FUNCTION_BLOCK FB 1004
TITLE =FB_SCTMi_IOL
//(*//////////////////////////////////////////////////////////////////////////////
////------------------------------------------------------------------------------
//// Copyright (C) - J. Schmalz GmbH 2018 - All Rights Reserved
//// Subject to change without notice
////------------------------------------------------------------------------------
//// This function block controls a Schmalz SCTMi with IO-Link interface via the
//// process data. With this function block all possible combinations of ejectors
//// can be controlled.
//// Further information can be found in the funktionblock documentation.
////------------------------------------------------------------------------------
//// Version:       1.0
//// Issue DATE:    2018-07-20
////------------------------------------------------------------------------------
////////////////////////////////////////////////////////////////////////////////*)

VERSION : 0.0


VAR_INPUT
  iInputPressure : INT ;
  bVacOnEjector1 : BOOL ;
  bBlowOffEjector1 : BOOL ;
  bVacOnEjector2 : BOOL ;
  bBlowOffEjector2 : BOOL ;
  bVacOnEjector3 : BOOL ;
  bBlowOffEjector3 : BOOL ;
  bVacOnEjector4 : BOOL ;
  bBlowOffEjector4 : BOOL ;
  bVacOnEjector5 : BOOL ;
  bBlowOffEjector5 : BOOL ;
  bVacOnEjector6 : BOOL ;
  bBlowOffEjector6 : BOOL ;
  bVacOnEjector7 : BOOL ;
  bBlowOffEjector7 : BOOL ;
  bVacOnEjector8 : BOOL ;
  bBlowOffEjector8 : BOOL ;
  bVacOnEjector9 : BOOL ;
  bBlowOffEjector9 : BOOL ;
  bVacOnEjector10 : BOOL ;
  bBlowOffEjector10 : BOOL ;
  bVacOnEjector11 : BOOL ;
  bBlowOffEjector11 : BOOL ;
  bVacOnEjector12 : BOOL ;
  bBlowOffEjector12 : BOOL ;
  bVacOnEjector13 : BOOL ;
  bBlowOffEjector13 : BOOL ;
  bVacOnEjector14 : BOOL ;
  bBlowOffEjector14 : BOOL ;
  bVacOnEjector15 : BOOL ;
  bBlowOffEjector15 : BOOL ;
  bVacOnEjector16 : BOOL ;
  bBlowOffEjector16 : BOOL ;
  iNumberOfEjectors : INT ;
  iValveTypes : INT ;
  btPDIData0 : BYTE ;
  btPDIData1 : BYTE ;
  btPDIData2 : BYTE ;
  btPDIData3 : BYTE ;
  btPDIData4 : BYTE ;
  btPDIData5 : BYTE ;
  btPDIData6 : BYTE ;
  btPDIData7 : BYTE ;
END_VAR
VAR_OUTPUT
  bDeviceStateGreen : BOOL ;
  bDeviceStateYellow : BOOL ;
  bDeviceStateOrange : BOOL ;
  bDeviceStateRed : BOOL ;
  btErrorByteCU : BYTE ;
  btWarningByteCU : BYTE ;
  wPrimSupplyVoltageCU : WORD ;
  wAuxSupplyVoltageCU : WORD ;
  wTotalAirConsCU : WORD ;
  stDataEjector1 : STRUCT
   btErrorByte : BYTE ;
   btWarningByte : BYTE ;
   btLeakageOfLastCycle : BYTE ;
   wSystemVacuum : WORD ;
   wEvacuationTimeT1 : WORD ;
   wLastFreeFlowVacuum : WORD ;
   wAirConsumptionOfLastCyc : WORD ;
   bAirSavingFunktion_H1 : BOOL ;
   bPartPresent_H2 : BOOL ;
  END_STRUCT ;
  stDataEjector2 : STRUCT
   btErrorByte : BYTE ;
   btWarningByte : BYTE ;
   btLeakageOfLastCycle : BYTE ;
   wSystemVacuum : WORD ;
   wEvacuationTimeT1 : WORD ;
   wLastFreeFlowVacuum : WORD ;
   wAirConsumptionOfLastCyc : WORD ;
   bAirSavingFunktion_H1 : BOOL ;
   bPartPresent_H2 : BOOL ;
  END_STRUCT ;
  stDataEjector3 : STRUCT
   btErrorByte : BYTE ;
   btWarningByte : BYTE ;
   btLeakageOfLastCycle : BYTE ;
   wSystemVacuum : WORD ;
   wEvacuationTimeT1 : WORD ;
   wLastFreeFlowVacuum : WORD ;
   wAirConsumptionOfLastCyc : WORD ;
   bAirSavingFunktion_H1 : BOOL ;
   bPartPresent_H2 : BOOL ;
  END_STRUCT ;
  stDataEjector4 : STRUCT
   btErrorByte : BYTE ;
   btWarningByte : BYTE ;
   btLeakageOfLastCycle : BYTE ;
   wSystemVacuum : WORD ;
   wEvacuationTimeT1 : WORD ;
   wLastFreeFlowVacuum : WORD ;
   wAirConsumptionOfLastCyc : WORD ;
   bAirSavingFunktion_H1 : BOOL ;
   bPartPresent_H2 : BOOL ;
  END_STRUCT ;
  stDataEjector5 : STRUCT
   btErrorByte : BYTE ;
   btWarningByte : BYTE ;
   btLeakageOfLastCycle : BYTE ;
   wSystemVacuum : WORD ;
   wEvacuationTimeT1 : WORD ;
   wLastFreeFlowVacuum : WORD ;
   wAirConsumptionOfLastCyc : WORD ;
   bAirSavingFunktion_H1 : BOOL ;
   bPartPresent_H2 : BOOL ;
  END_STRUCT ;
  stDataEjector6 : STRUCT
   btErrorByte : BYTE ;
   btWarningByte : BYTE ;
   btLeakageOfLastCycle : BYTE ;
   wSystemVacuum : WORD ;
   wEvacuationTimeT1 : WORD ;
   wLastFreeFlowVacuum : WORD ;
   wAirConsumptionOfLastCyc : WORD ;
   bAirSavingFunktion_H1 : BOOL ;
   bPartPresent_H2 : BOOL ;
  END_STRUCT ;
  stDataEjector7 : STRUCT
   btErrorByte : BYTE ;
   btWarningByte : BYTE ;
   btLeakageOfLastCycle : BYTE ;
   wSystemVacuum : WORD ;
   wEvacuationTimeT1 : WORD ;
   wLastFreeFlowVacuum : WORD ;
   wAirConsumptionOfLastCyc : WORD ;
   bAirSavingFunktion_H1 : BOOL ;
   bPartPresent_H2 : BOOL ;
  END_STRUCT ;
  stDataEjector8 : STRUCT
   btErrorByte : BYTE ;
   btWarningByte : BYTE ;
   btLeakageOfLastCycle : BYTE ;
   wSystemVacuum : WORD ;
   wEvacuationTimeT1 : WORD ;
   wLastFreeFlowVacuum : WORD ;
   wAirConsumptionOfLastCyc : WORD ;
   bAirSavingFunktion_H1 : BOOL ;
   bPartPresent_H2 : BOOL ;
  END_STRUCT ;
  stDataEjector9 : STRUCT
   btErrorByte : BYTE ;
   btWarningByte : BYTE ;
   btLeakageOfLastCycle : BYTE ;
   wSystemVacuum : WORD ;
   wEvacuationTimeT1 : WORD ;
   wLastFreeFlowVacuum : WORD ;
   wAirConsumptionOfLastCyc : WORD ;
   bAirSavingFunktion_H1 : BOOL ;
   bPartPresent_H2 : BOOL ;
  END_STRUCT ;
  stDataEjector10 : STRUCT
   btErrorByte : BYTE ;
   btWarningByte : BYTE ;
   btLeakageOfLastCycle : BYTE ;
   wSystemVacuum : WORD ;
   wEvacuationTimeT1 : WORD ;
   wLastFreeFlowVacuum : WORD ;
   wAirConsumptionOfLastCyc : WORD ;
   bAirSavingFunktion_H1 : BOOL ;
   bPartPresent_H2 : BOOL ;
  END_STRUCT ;
  stDataEjector11 : STRUCT
   btErrorByte : BYTE ;
   btWarningByte : BYTE ;
   btLeakageOfLastCycle : BYTE ;
   wSystemVacuum : WORD ;
   wEvacuationTimeT1 : WORD ;
   wLastFreeFlowVacuum : WORD ;
   wAirConsumptionOfLastCyc : WORD ;
   bAirSavingFunktion_H1 : BOOL ;
   bPartPresent_H2 : BOOL ;
  END_STRUCT ;
  stDataEjector12 : STRUCT
   btErrorByte : BYTE ;
   btWarningByte : BYTE ;
   btLeakageOfLastCycle : BYTE ;
   wSystemVacuum : WORD ;
   wEvacuationTimeT1 : WORD ;
   wLastFreeFlowVacuum : WORD ;
   wAirConsumptionOfLastCyc : WORD ;
   bAirSavingFunktion_H1 : BOOL ;
   bPartPresent_H2 : BOOL ;
  END_STRUCT ;
  stDataEjector13 : STRUCT
   btErrorByte : BYTE ;
   btWarningByte : BYTE ;
   btLeakageOfLastCycle : BYTE ;
   wSystemVacuum : WORD ;
   wEvacuationTimeT1 : WORD ;
   wLastFreeFlowVacuum : WORD ;
   wAirConsumptionOfLastCyc : WORD ;
   bAirSavingFunktion_H1 : BOOL ;
   bPartPresent_H2 : BOOL ;
  END_STRUCT ;
  stDataEjector14 : STRUCT
   btErrorByte : BYTE ;
   btWarningByte : BYTE ;
   btLeakageOfLastCycle : BYTE ;
   wSystemVacuum : WORD ;
   wEvacuationTimeT1 : WORD ;
   wLastFreeFlowVacuum : WORD ;
   wAirConsumptionOfLastCyc : WORD ;
   bAirSavingFunktion_H1 : BOOL ;
   bPartPresent_H2 : BOOL ;
  END_STRUCT ;
  stDataEjector15 : STRUCT
   btErrorByte : BYTE ;
   btWarningByte : BYTE ;
   btLeakageOfLastCycle : BYTE ;
   wSystemVacuum : WORD ;
   wEvacuationTimeT1 : WORD ;
   wLastFreeFlowVacuum : WORD ;
   wAirConsumptionOfLastCyc : WORD ;
   bAirSavingFunktion_H1 : BOOL ;
   bPartPresent_H2 : BOOL ;
  END_STRUCT ;
  stDataEjector16 : STRUCT
   btErrorByte : BYTE ;
   btWarningByte : BYTE ;
   btLeakageOfLastCycle : BYTE ;
   wSystemVacuum : WORD ;
   wEvacuationTimeT1 : WORD ;
   wLastFreeFlowVacuum : WORD ;
   wAirConsumptionOfLastCyc : WORD ;
   bAirSavingFunktion_H1 : BOOL ;
   bPartPresent_H2 : BOOL ;
  END_STRUCT ;
  btPDOData0 : BYTE ;
  btPDOData1 : BYTE ;
  btPDOData2 : BYTE ;
  btPDOData3 : BYTE ;
  btPDOData4 : BYTE ;
  btPDOData5 : BYTE ;
END_VAR
VAR
  iStep : INT ;
END_VAR
BEGIN
NETWORK
TITLE =SCL Netzwerk
//generiert vom SCL Übersetzer Version:  SCLCOMP K05.06.00.00_11.01.00.01 release
      SET   ;
      SAVE  ;
      =     L      0.1;
      L     #iStep;
      L     0;
      TAK   ;
      ==I   ;
      T     LW     2;
      SPB   A7d1;
      SPA   A7d2;
A7d1: CLR   ;
      =     DIX [AR2,P#252.0];
      =     DIX [AR2,P#252.1];
      =     DIX [AR2,P#252.2];
      =     DIX [AR2,P#252.3];
      =     DIX [AR2,P#252.4];
      =     DIX [AR2,P#252.6];
      =     DIX [AR2,P#252.7];
      U     DIX [AR2,P#10.5];
      NOT   ;
      SPBN  A7d0;
      L     #btPDIData1;
      T     #btErrorByteCU;
      L     #btPDIData3;
      T     DIB [AR2,P#22.0];
      L     #btPDIData2;
      T     DIB [AR2,P#23.0];
      L     #iStep;
      L     1;
      +I    ;
      T     #iStep;
      SPA   A7d0;
A7d2: L     1;
      L     LW     2;
      ==I   ;
      SPB   A7d4;
      SPA   A7d5;
A7d4: SET   ;
      =     DIX [AR2,P#252.6];
      CLR   ;
      =     DIX [AR2,P#252.7];
      U     DIX [AR2,P#10.5];
      SPBN  A7d0;
      L     #btPDIData1;
      T     #btWarningByteCU;
      L     #btPDIData3;
      T     DIB [AR2,P#24.0];
      L     #btPDIData2;
      T     DIB [AR2,P#25.0];
      L     #iStep;
      L     1;
      +I    ;
      T     #iStep;
      SPA   A7d0;
A7d5: L     2;
      L     LW     2;
      ==I   ;
      SPB   A7d7;
      SPA   A7d8;
A7d7: CLR   ;
      =     DIX [AR2,P#252.6];
      =     DIX [AR2,P#252.7];
      U     DIX [AR2,P#10.5];
      NOT   ;
      SPBN  A7d0;
      L     #iStep;
      L     1;
      +I    ;
      T     #iStep;
      SPA   A7d0;
A7d8: L     3;
      L     LW     2;
      ==I   ;
      SPB   A7da;
      SPA   A7db;
A7da: CLR   ;
      =     DIX [AR2,P#252.6];
      SET   ;
      =     DIX [AR2,P#252.7];
      U     DIX [AR2,P#10.5];
      SPBN  A7d0;
      L     #iStep;
      L     1;
      +I    ;
      T     #iStep;
      SPA   A7d0;
A7db: L     4;
      L     LW     2;
      ==I   ;
      SPB   A7dd;
      SPA   A7de;
A7dd: CLR   ;
      =     DIX [AR2,P#252.6];
      =     DIX [AR2,P#252.7];
      U     DIX [AR2,P#10.5];
      NOT   ;
      SPBN  A7d0;
      L     #iStep;
      L     1;
      +I    ;
      T     #iStep;
      SPA   A7d0;
A7de: L     5;
      L     LW     2;
      ==I   ;
      SPB   A7e0;
      SPA   A7e1;
A7e0: SET   ;
      =     DIX [AR2,P#252.6];
      =     DIX [AR2,P#252.7];
      U     DIX [AR2,P#10.5];
      SPBN  A7d0;
      L     #btPDIData3;
      T     DIB [AR2,P#26.0];
      L     #btPDIData2;
      T     DIB [AR2,P#27.0];
      L     #iStep;
      L     1;
      +I    ;
      T     #iStep;
      SPA   A7d0;
A7e1: L     6;
      L     LW     2;
      ==I   ;
      SPB   A7e3;
      SPA   A7e4;
A7e3: L     #iNumberOfEjectors;
      L     1;
      >=I   ;
      SPBN  A7e5;
      L     #iStep;
      +I    ;
      T     #iStep;
      SPA   A7d0;
A7e5: L     0;
      T     #iStep;
      SPA   A7d0;
A7e4: L     7;
      L     LW     2;
      ==I   ;
      SPB   A7e7;
      SPA   A7e8;
A7e7: SET   ;
      =     DIX [AR2,P#252.0];
      CLR   ;
      =     DIX [AR2,P#252.1];
      =     DIX [AR2,P#252.2];
      =     DIX [AR2,P#252.3];
      =     DIX [AR2,P#252.4];
      =     DIX [AR2,P#252.6];
      =     DIX [AR2,P#252.7];
      U     DIX [AR2,P#10.5];
      NOT   ;
      SPBN  A7d0;
      L     #btPDIData1;
      T     #stDataEjector1.btErrorByte;
      L     #btPDIData2;
      UD    DW#16#FF;
      L     8;
      TAK   ;
      LAR1  ;
      TAK   ;
      L     DW#16#10;
      >=I   ;
      SPB   I007;
      TAK   ;
      TAR1  ;
      SLW   ;
      SPA   I008;
I007: L     DW#16#0;
I008: UD    DW#16#FFFF;
      L     #btPDIData3;
      UD    DW#16#FF;
      OW    ;
      T     #stDataEjector1.wSystemVacuum;
      L     #iStep;
      L     1;
      +I    ;
      T     #iStep;
      SPA   A7d0;
A7e8: L     8;
      L     LW     2;
      ==I   ;
      SPB   A7ea;
      SPA   A7eb;
A7ea: SET   ;
      =     DIX [AR2,P#252.6];
      CLR   ;
      =     DIX [AR2,P#252.7];
      U     DIX [AR2,P#10.5];
      SPBN  A7d0;
      L     #btPDIData1;
      T     #stDataEjector1.btWarningByte;
      L     #btPDIData2;
      UD    DW#16#FF;
      L     8;
      TAK   ;
      LAR1  ;
      TAK   ;
      L     DW#16#10;
      >=I   ;
      SPB   I009;
      TAK   ;
      TAR1  ;
      SLW   ;
      SPA   I00a;
I009: L     DW#16#0;
I00a: UD    DW#16#FFFF;
      L     #btPDIData3;
      UD    DW#16#FF;
      OW    ;
      T     #stDataEjector1.wEvacuationTimeT1;
      L     #iStep;
      L     1;
      +I    ;
      T     #iStep;
      SPA   A7d0;
A7eb: L     9;
      L     LW     2;
      ==I   ;
      SPB   A7ed;
      SPA   A7ee;
A7ed: CLR   ;
      =     DIX [AR2,P#252.6];
      =     DIX [AR2,P#252.7];
      U     DIX [AR2,P#10.5];
      NOT   ;
      SPBN  A7d0;
      L     #iStep;
      L     1;
      +I    ;
      T     #iStep;
      SPA   A7d0;
A7ee: L     10;
      L     LW     2;
      ==I   ;
      SPB   A7f0;
      SPA   A7f1;
A7f0: CLR   ;
      =     DIX [AR2,P#252.6];
      SET   ;
      =     DIX [AR2,P#252.7];
      U     DIX [AR2,P#10.5];
      SPBN  A7d0;
      L     #btPDIData2;
      UD    DW#16#FF;
      L     8;
      TAK   ;
      LAR1  ;
      TAK   ;
      L     DW#16#10;
      >=I   ;
      SPB   I00b;
      TAK   ;
      TAR1  ;
      SLW   ;
      SPA   I00c;
I00b: L     DW#16#0;
I00c: UD    DW#16#FFFF;
      L     #btPDIData3;
      UD    DW#16#FF;
      OW    ;
      T     #stDataEjector1.wLastFreeFlowVacuum;
      L     #iStep;
      L     1;
      +I    ;
      T     #iStep;
      SPA   A7d0;
A7f1: L     11;
      L     LW     2;
      ==I   ;
      SPB   A7f3;
      SPA   A7f4;
A7f3: CLR   ;
      =     DIX [AR2,P#252.6];
      =     DIX [AR2,P#252.7];
      U     DIX [AR2,P#10.5];
      NOT   ;
      SPBN  A7d0;
      L     #iStep;
      L     1;
      +I    ;
      T     #iStep;
      SPA   A7d0;
A7f4: L     12;
      L     LW     2;
      ==I   ;
      SPB   A7f6;
      SPA   A7f7;
A7f6: SET   ;
      =     DIX [AR2,P#252.6];
      =     DIX [AR2,P#252.7];
      U     DIX [AR2,P#10.5];
      SPBN  A7d0;
      L     #btPDIData1;
      T     #stDataEjector1.btLeakageOfLastCycle;
      L     #btPDIData2;
      UD    DW#16#FF;
      L     8;
      TAK   ;
      LAR1  ;
      TAK   ;
      L     DW#16#10;
      >=I   ;
      SPB   I00d;
      TAK   ;
      TAR1  ;
      SLW   ;
      SPA   I00e;
I00d: L     DW#16#0;
I00e: UD    DW#16#FFFF;
      L     #btPDIData3;
      UD    DW#16#FF;
      OW    ;
      T     #stDataEjector1.wAirConsumptionOfLastCyc;
      L     #iStep;
      L     1;
      +I    ;
      T     #iStep;
      SPA   A7d0;
A7f7: L     13;
      L     LW     2;
      ==I   ;
      SPB   A7f9;
      SPA   A7fa;
A7f9: L     #iNumberOfEjectors;
      L     2;
      >=I   ;
      SPBN  A7fb;
      L     #iStep;
      L     1;
      +I    ;
      T     #iStep;
      SPA   A7d0;
A7fb: L     0;
      T     #iStep;
      SPA   A7d0;
A7fa: L     14;
      L     LW     2;
      ==I   ;
      SPB   A7fd;
      SPA   A7fe;
A7fd: CLR   ;
      =     DIX [AR2,P#252.0];
      SET   ;
      =     DIX [AR2,P#252.1];
      CLR   ;
      =     DIX [AR2,P#252.2];
      =     DIX [AR2,P#252.3];
      =     DIX [AR2,P#252.4];
      =     DIX [AR2,P#252.6];
      =     DIX [AR2,P#252.7];
      U     DIX [AR2,P#10.5];
      NOT   ;
      SPBN  A7d0;
      L     #btPDIData1;
      T     #stDataEjector2.btErrorByte;
      L     #btPDIData2;
      UD    DW#16#FF;
      L     8;
      TAK   ;
      LAR1  ;
      TAK   ;
      L     DW#16#10;
      >=I   ;
      SPB   I00f;
      TAK   ;
      TAR1  ;
      SLW   ;
      SPA   I010;
I00f: L     DW#16#0;
I010: UD    DW#16#FFFF;
      L     #btPDIData3;
      UD    DW#16#FF;
      OW    ;
      T     #stDataEjector2.wSystemVacuum;
      L     #iStep;
      L     1;
      +I    ;
      T     #iStep;
      SPA   A7d0;
A7fe: L     15;
      L     LW     2;
      ==I   ;
      SPB   A800;
      SPA   A801;
A800: SET   ;
      =     DIX [AR2,P#252.6];
      CLR   ;
      =     DIX [AR2,P#252.7];
      U     DIX [AR2,P#10.5];
      SPBN  A7d0;
      L     #btPDIData1;
      T     #stDataEjector2.btWarningByte;
      L     #btPDIData2;
      UD    DW#16#FF;
      L     8;
      TAK   ;
      LAR1  ;
      TAK   ;
      L     DW#16#10;
      >=I   ;
      SPB   I011;
      TAK   ;
      TAR1  ;
      SLW   ;
      SPA   I012;
I011: L     DW#16#0;
I012: UD    DW#16#FFFF;
      L     #btPDIData3;
      UD    DW#16#FF;
      OW    ;
      T     #stDataEjector2.wEvacuationTimeT1;
      L     #iStep;
      L     1;
      +I    ;
      T     #iStep;
      SPA   A7d0;
A801: L     16;
      L     LW     2;
      ==I   ;
      SPB   A803;
      SPA   A804;
A803: CLR   ;
      =     DIX [AR2,P#252.6];
      =     DIX [AR2,P#252.7];
      U     DIX [AR2,P#10.5];
      NOT   ;
      SPBN  A7d0;
      L     #iStep;
      L     1;
      +I    ;
      T     #iStep;
      SPA   A7d0;
A804: L     17;
      L     LW     2;
      ==I   ;
      SPB   A806;
      SPA   A807;
A806: CLR   ;
      =     DIX [AR2,P#252.6];
      SET   ;
      =     DIX [AR2,P#252.7];
      U     DIX [AR2,P#10.5];
      SPBN  A7d0;
      L     #btPDIData2;
      UD    DW#16#FF;
      L     8;
      TAK   ;
      LAR1  ;
      TAK   ;
      L     DW#16#10;
      >=I   ;
      SPB   I013;
      TAK   ;
      TAR1  ;
      SLW   ;
      SPA   I014;
I013: L     DW#16#0;
I014: UD    DW#16#FFFF;
      L     #btPDIData3;
      UD    DW#16#FF;
      OW    ;
      T     #stDataEjector2.wLastFreeFlowVacuum;
      L     #iStep;
      L     1;
      +I    ;
      T     #iStep;
      SPA   A7d0;
A807: L     18;
      L     LW     2;
      ==I   ;
      SPB   A809;
      SPA   A80a;
A809: CLR   ;
      =     DIX [AR2,P#252.6];
      =     DIX [AR2,P#252.7];
      U     DIX [AR2,P#10.5];
      NOT   ;
      SPBN  A7d0;
      L     #iStep;
      L     1;
      +I    ;
      T     #iStep;
      SPA   A7d0;
A80a: L     19;
      L     LW     2;
      ==I   ;
      SPB   A80c;
      SPA   A80d;
A80c: SET   ;
      =     DIX [AR2,P#252.6];
      =     DIX [AR2,P#252.7];
      U     DIX [AR2,P#10.5];
      SPBN  A7d0;
      L     #btPDIData1;
      T     #stDataEjector2.btLeakageOfLastCycle;
      L     #btPDIData2;
      UD    DW#16#FF;
      L     8;
      TAK   ;
      LAR1  ;
      TAK   ;
      L     DW#16#10;
      >=I   ;
      SPB   I015;
      TAK   ;
      TAR1  ;
      SLW   ;
      SPA   I016;
I015: L     DW#16#0;
I016: UD    DW#16#FFFF;
      L     #btPDIData3;
      UD    DW#16#FF;
      OW    ;
      T     #stDataEjector2.wAirConsumptionOfLastCyc;
      L     #iStep;
      L     1;
      +I    ;
      T     #iStep;
      SPA   A7d0;
A80d: L     20;
      L     LW     2;
      ==I   ;
      SPB   A80f;
      SPA   A810;
A80f: L     #iNumberOfEjectors;
      L     3;
      >=I   ;
      SPBN  A811;
      L     #iStep;
      L     1;
      +I    ;
      T     #iStep;
      SPA   A7d0;
A811: L     0;
      T     #iStep;
      SPA   A7d0;
A810: L     21;
      L     LW     2;
      ==I   ;
      SPB   A813;
      SPA   A814;
A813: SET   ;
      =     DIX [AR2,P#252.0];
      =     DIX [AR2,P#252.1];
      CLR   ;
      =     DIX [AR2,P#252.2];
      =     DIX [AR2,P#252.3];
      =     DIX [AR2,P#252.4];
      =     DIX [AR2,P#252.6];
      =     DIX [AR2,P#252.7];
      U     DIX [AR2,P#10.5];
      NOT   ;
      SPBN  A7d0;
      L     #btPDIData1;
      T     #stDataEjector3.btErrorByte;
      L     #btPDIData2;
      UD    DW#16#FF;
      L     8;
      TAK   ;
      LAR1  ;
      TAK   ;
      L     DW#16#10;
      >=I   ;
      SPB   I017;
      TAK   ;
      TAR1  ;
      SLW   ;
      SPA   I018;
I017: L     DW#16#0;
I018: UD    DW#16#FFFF;
      L     #btPDIData3;
      UD    DW#16#FF;
      OW    ;
      T     #stDataEjector3.wSystemVacuum;
      L     #iStep;
      L     1;
      +I    ;
      T     #iStep;
      SPA   A7d0;
A814: L     22;
      L     LW     2;
      ==I   ;
      SPB   A816;
      SPA   A817;
A816: SET   ;
      =     DIX [AR2,P#252.6];
      CLR   ;
      =     DIX [AR2,P#252.7];
      U     DIX [AR2,P#10.5];
      SPBN  A7d0;
      L     #btPDIData1;
      T     #stDataEjector3.btWarningByte;
      L     #btPDIData2;
      UD    DW#16#FF;
      L     8;
      TAK   ;
      LAR1  ;
      TAK   ;
      L     DW#16#10;
      >=I   ;
      SPB   I019;
      TAK   ;
      TAR1  ;
      SLW   ;
      SPA   I01a;
I019: L     DW#16#0;
I01a: UD    DW#16#FFFF;
      L     #btPDIData3;
      UD    DW#16#FF;
      OW    ;
      T     #stDataEjector3.wEvacuationTimeT1;
      L     #iStep;
      L     1;
      +I    ;
      T     #iStep;
      SPA   A7d0;
A817: L     23;
      L     LW     2;
      ==I   ;
      SPB   A819;
      SPA   A81a;
A819: CLR   ;
      =     DIX [AR2,P#252.6];
      =     DIX [AR2,P#252.7];
      U     DIX [AR2,P#10.5];
      NOT   ;
      SPBN  A7d0;
      L     #iStep;
      L     1;
      +I    ;
      T     #iStep;
      SPA   A7d0;
A81a: L     24;
      L     LW     2;
      ==I   ;
      SPB   A81c;
      SPA   A81d;
A81c: CLR   ;
      =     DIX [AR2,P#252.6];
      SET   ;
      =     DIX [AR2,P#252.7];
      U     DIX [AR2,P#10.5];
      SPBN  A7d0;
      L     #btPDIData2;
      UD    DW#16#FF;
      L     8;
      TAK   ;
      LAR1  ;
      TAK   ;
      L     DW#16#10;
      >=I   ;
      SPB   I01b;
      TAK   ;
      TAR1  ;
      SLW   ;
      SPA   I01c;
I01b: L     DW#16#0;
I01c: UD    DW#16#FFFF;
      L     #btPDIData3;
      UD    DW#16#FF;
      OW    ;
      T     #stDataEjector3.wLastFreeFlowVacuum;
      L     #iStep;
      L     1;
      +I    ;
      T     #iStep;
      SPA   A7d0;
A81d: L     25;
      L     LW     2;
      ==I   ;
      SPB   A81f;
      SPA   A820;
A81f: CLR   ;
      =     DIX [AR2,P#252.6];
      =     DIX [AR2,P#252.7];
      U     DIX [AR2,P#10.5];
      NOT   ;
      SPBN  A7d0;
      L     #iStep;
      L     1;
      +I    ;
      T     #iStep;
      SPA   A7d0;
A820: L     26;
      L     LW     2;
      ==I   ;
      SPB   A822;
      SPA   A823;
A822: SET   ;
      =     DIX [AR2,P#252.6];
      =     DIX [AR2,P#252.7];
      U     DIX [AR2,P#10.5];
      SPBN  A7d0;
      L     #btPDIData1;
      T     #stDataEjector3.btLeakageOfLastCycle;
      L     #btPDIData2;
      UD    DW#16#FF;
      L     8;
      TAK   ;
      LAR1  ;
      TAK   ;
      L     DW#16#10;
      >=I   ;
      SPB   I01d;
      TAK   ;
      TAR1  ;
      SLW   ;
      SPA   I01e;
I01d: L     DW#16#0;
I01e: UD    DW#16#FFFF;
      L     #btPDIData3;
      UD    DW#16#FF;
      OW    ;
      T     #stDataEjector3.wAirConsumptionOfLastCyc;
      L     #iStep;
      L     1;
      +I    ;
      T     #iStep;
      SPA   A7d0;
A823: L     27;
      L     LW     2;
      ==I   ;
      SPB   A825;
      SPA   A826;
A825: L     #iNumberOfEjectors;
      L     4;
      >=I   ;
      SPBN  A827;
      L     #iStep;
      L     1;
      +I    ;
      T     #iStep;
      SPA   A7d0;
A827: L     0;
      T     #iStep;
      SPA   A7d0;
A826: L     28;
      L     LW     2;
      ==I   ;
      SPB   A829;
      SPA   A82a;
A829: CLR   ;
      =     DIX [AR2,P#252.0];
      =     DIX [AR2,P#252.1];
      SET   ;
      =     DIX [AR2,P#252.2];
      CLR   ;
      =     DIX [AR2,P#252.3];
      =     DIX [AR2,P#252.4];
      =     DIX [AR2,P#252.6];
      =     DIX [AR2,P#252.7];
      U     DIX [AR2,P#10.5];
      NOT   ;
      SPBN  A7d0;
      L     #btPDIData1;
      T     #stDataEjector4.btErrorByte;
      L     #btPDIData2;
      UD    DW#16#FF;
      L     8;
      TAK   ;
      LAR1  ;
      TAK   ;
      L     DW#16#10;
      >=I   ;
      SPB   I01f;
      TAK   ;
      TAR1  ;
      SLW   ;
      SPA   I020;
I01f: L     DW#16#0;
I020: UD    DW#16#FFFF;
      L     #btPDIData3;
      UD    DW#16#FF;
      OW    ;
      T     #stDataEjector4.wSystemVacuum;
      L     #iStep;
      L     1;
      +I    ;
      T     #iStep;
      SPA   A7d0;
A82a: L     29;
      L     LW     2;
      ==I   ;
      SPB   A82c;
      SPA   A82d;
A82c: SET   ;
      =     DIX [AR2,P#252.6];
      CLR   ;
      =     DIX [AR2,P#252.7];
      U     DIX [AR2,P#10.5];
      SPBN  A7d0;
      L     #btPDIData1;
      T     #stDataEjector4.btWarningByte;
      L     #btPDIData2;
      UD    DW#16#FF;
      L     8;
      TAK   ;
      LAR1  ;
      TAK   ;
      L     DW#16#10;
      >=I   ;
      SPB   I021;
      TAK   ;
      TAR1  ;
      SLW   ;
      SPA   I022;
I021: L     DW#16#0;
I022: UD    DW#16#FFFF;
      L     #btPDIData3;
      UD    DW#16#FF;
      OW    ;
      T     #stDataEjector4.wEvacuationTimeT1;
      L     #iStep;
      L     1;
      +I    ;
      T     #iStep;
      SPA   A7d0;
A82d: L     30;
      L     LW     2;
      ==I   ;
      SPB   A82f;
      SPA   A830;
A82f: CLR   ;
      =     DIX [AR2,P#252.6];
      =     DIX [AR2,P#252.7];
      U     DIX [AR2,P#10.5];
      NOT   ;
      SPBN  A7d0;
      L     #iStep;
      L     1;
      +I    ;
      T     #iStep;
      SPA   A7d0;
A830: L     31;
      L     LW     2;
      ==I   ;
      SPB   A832;
      SPA   A833;
A832: CLR   ;
      =     DIX [AR2,P#252.6];
      SET   ;
      =     DIX [AR2,P#252.7];
      U     DIX [AR2,P#10.5];
      SPBN  A7d0;
      L     #btPDIData2;
      UD    DW#16#FF;
      L     8;
      TAK   ;
      LAR1  ;
      TAK   ;
      L     DW#16#10;
      >=I   ;
      SPB   I023;
      TAK   ;
      TAR1  ;
      SLW   ;
      SPA   I024;
I023: L     DW#16#0;
I024: UD    DW#16#FFFF;
      L     #btPDIData3;
      UD    DW#16#FF;
      OW    ;
      T     #stDataEjector4.wLastFreeFlowVacuum;
      L     #iStep;
      L     1;
      +I    ;
      T     #iStep;
      SPA   A7d0;
A833: L     32;
      L     LW     2;
      ==I   ;
      SPB   A835;
      SPA   A836;
A835: CLR   ;
      =     DIX [AR2,P#252.6];
      =     DIX [AR2,P#252.7];
      U     DIX [AR2,P#10.5];
      NOT   ;
      SPBN  A7d0;
      L     #iStep;
      L     1;
      +I    ;
      T     #iStep;
      SPA   A7d0;
A836: L     33;
      L     LW     2;
      ==I   ;
      SPB   A838;
      SPA   A839;
A838: SET   ;
      =     DIX [AR2,P#252.6];
      =     DIX [AR2,P#252.7];
      U     DIX [AR2,P#10.5];
      SPBN  A7d0;
      L     #btPDIData1;
      T     #stDataEjector4.btLeakageOfLastCycle;
      L     #btPDIData2;
      UD    DW#16#FF;
      L     8;
      TAK   ;
      LAR1  ;
      TAK   ;
      L     DW#16#10;
      >=I   ;
      SPB   I025;
      TAK   ;
      TAR1  ;
      SLW   ;
      SPA   I026;
I025: L     DW#16#0;
I026: UD    DW#16#FFFF;
      L     #btPDIData3;
      UD    DW#16#FF;
      OW    ;
      T     #stDataEjector4.wAirConsumptionOfLastCyc;
      L     #iStep;
      L     1;
      +I    ;
      T     #iStep;
      SPA   A7d0;
A839: L     34;
      L     LW     2;
      ==I   ;
      SPB   A83b;
      SPA   A83c;
A83b: L     #iNumberOfEjectors;
      L     5;
      >=I   ;
      SPBN  A83d;
      L     #iStep;
      L     1;
      +I    ;
      T     #iStep;
      SPA   A7d0;
A83d: L     0;
      T     #iStep;
      SPA   A7d0;
A83c: L     35;
      L     LW     2;
      ==I   ;
      SPB   A83f;
      SPA   A840;
A83f: SET   ;
      =     DIX [AR2,P#252.0];
      CLR   ;
      =     DIX [AR2,P#252.1];
      SET   ;
      =     DIX [AR2,P#252.2];
      CLR   ;
      =     DIX [AR2,P#252.3];
      =     DIX [AR2,P#252.4];
      =     DIX [AR2,P#252.6];
      =     DIX [AR2,P#252.7];
      U     DIX [AR2,P#10.5];
      NOT   ;
      SPBN  A7d0;
      L     #btPDIData1;
      T     #stDataEjector5.btErrorByte;
      L     #btPDIData2;
      UD    DW#16#FF;
      L     8;
      TAK   ;
      LAR1  ;
      TAK   ;
      L     DW#16#10;
      >=I   ;
      SPB   I027;
      TAK   ;
      TAR1  ;
      SLW   ;
      SPA   I028;
I027: L     DW#16#0;
I028: UD    DW#16#FFFF;
      L     #btPDIData3;
      UD    DW#16#FF;
      OW    ;
      T     #stDataEjector5.wSystemVacuum;
      L     #iStep;
      L     1;
      +I    ;
      T     #iStep;
      SPA   A7d0;
A840: L     36;
      L     LW     2;
      ==I   ;
      SPB   A842;
      SPA   A843;
A842: SET   ;
      =     DIX [AR2,P#252.6];
      CLR   ;
      =     DIX [AR2,P#252.7];
      U     DIX [AR2,P#10.5];
      SPBN  A7d0;
      L     #btPDIData1;
      T     #stDataEjector5.btWarningByte;
      L     #btPDIData2;
      UD    DW#16#FF;
      L     8;
      TAK   ;
      LAR1  ;
      TAK   ;
      L     DW#16#10;
      >=I   ;
      SPB   I029;
      TAK   ;
      TAR1  ;
      SLW   ;
      SPA   I02a;
I029: L     DW#16#0;
I02a: UD    DW#16#FFFF;
      L     #btPDIData3;
      UD    DW#16#FF;
      OW    ;
      T     #stDataEjector5.wEvacuationTimeT1;
      L     #iStep;
      L     1;
      +I    ;
      T     #iStep;
      SPA   A7d0;
A843: L     37;
      L     LW     2;
      ==I   ;
      SPB   A845;
      SPA   A846;
A845: CLR   ;
      =     DIX [AR2,P#252.6];
      =     DIX [AR2,P#252.7];
      U     DIX [AR2,P#10.5];
      NOT   ;
      SPBN  A7d0;
      L     #iStep;
      L     1;
      +I    ;
      T     #iStep;
      SPA   A7d0;
A846: L     38;
      L     LW     2;
      ==I   ;
      SPB   A848;
      SPA   A849;
A848: CLR   ;
      =     DIX [AR2,P#252.6];
      SET   ;
      =     DIX [AR2,P#252.7];
      U     DIX [AR2,P#10.5];
      SPBN  A7d0;
      L     #btPDIData2;
      UD    DW#16#FF;
      L     8;
      TAK   ;
      LAR1  ;
      TAK   ;
      L     DW#16#10;
      >=I   ;
      SPB   I02b;
      TAK   ;
      TAR1  ;
      SLW   ;
      SPA   I02c;
I02b: L     DW#16#0;
I02c: UD    DW#16#FFFF;
      L     #btPDIData3;
      UD    DW#16#FF;
      OW    ;
      T     #stDataEjector5.wLastFreeFlowVacuum;
      L     #iStep;
      L     1;
      +I    ;
      T     #iStep;
      SPA   A7d0;
A849: L     39;
      L     LW     2;
      ==I   ;
      SPB   A84b;
      SPA   A84c;
A84b: CLR   ;
      =     DIX [AR2,P#252.6];
      =     DIX [AR2,P#252.7];
      U     DIX [AR2,P#10.5];
      NOT   ;
      SPBN  A7d0;
      L     #iStep;
      L     1;
      +I    ;
      T     #iStep;
      SPA   A7d0;
A84c: L     40;
      L     LW     2;
      ==I   ;
      SPB   A84e;
      SPA   A84f;
A84e: SET   ;
      =     DIX [AR2,P#252.6];
      =     DIX [AR2,P#252.7];
      U     DIX [AR2,P#10.5];
      SPBN  A7d0;
      L     #btPDIData1;
      T     #stDataEjector5.btLeakageOfLastCycle;
      L     #btPDIData2;
      UD    DW#16#FF;
      L     8;
      TAK   ;
      LAR1  ;
      TAK   ;
      L     DW#16#10;
      >=I   ;
      SPB   I02d;
      TAK   ;
      TAR1  ;
      SLW   ;
      SPA   I02e;
I02d: L     DW#16#0;
I02e: UD    DW#16#FFFF;
      L     #btPDIData3;
      UD    DW#16#FF;
      OW    ;
      T     #stDataEjector5.wAirConsumptionOfLastCyc;
      L     #iStep;
      L     1;
      +I    ;
      T     #iStep;
      SPA   A7d0;
A84f: L     41;
      L     LW     2;
      ==I   ;
      SPB   A851;
      SPA   A852;
A851: L     #iNumberOfEjectors;
      L     6;
      >=I   ;
      SPBN  A853;
      L     #iStep;
      L     1;
      +I    ;
      T     #iStep;
      SPA   A7d0;
A853: L     0;
      T     #iStep;
      SPA   A7d0;
A852: L     42;
      L     LW     2;
      ==I   ;
      SPB   A855;
      SPA   A856;
A855: CLR   ;
      =     DIX [AR2,P#252.0];
      SET   ;
      =     DIX [AR2,P#252.1];
      =     DIX [AR2,P#252.2];
      CLR   ;
      =     DIX [AR2,P#252.3];
      =     DIX [AR2,P#252.4];
      =     DIX [AR2,P#252.6];
      =     DIX [AR2,P#252.7];
      U     DIX [AR2,P#10.5];
      NOT   ;
      SPBN  A7d0;
      L     #btPDIData1;
      T     #stDataEjector6.btErrorByte;
      L     #btPDIData2;
      UD    DW#16#FF;
      L     8;
      TAK   ;
      LAR1  ;
      TAK   ;
      L     DW#16#10;
      >=I   ;
      SPB   I02f;
      TAK   ;
      TAR1  ;
      SLW   ;
      SPA   I030;
I02f: L     DW#16#0;
I030: UD    DW#16#FFFF;
      L     #btPDIData3;
      UD    DW#16#FF;
      OW    ;
      T     #stDataEjector6.wSystemVacuum;
      L     #iStep;
      L     1;
      +I    ;
      T     #iStep;
      SPA   A7d0;
A856: L     43;
      L     LW     2;
      ==I   ;
      SPB   A858;
      SPA   A859;
A858: SET   ;
      =     DIX [AR2,P#252.6];
      CLR   ;
      =     DIX [AR2,P#252.7];
      U     DIX [AR2,P#10.5];
      SPBN  A7d0;
      L     #btPDIData1;
      T     #stDataEjector6.btWarningByte;
      L     #btPDIData2;
      UD    DW#16#FF;
      L     8;
      TAK   ;
      LAR1  ;
      TAK   ;
      L     DW#16#10;
      >=I   ;
      SPB   I031;
      TAK   ;
      TAR1  ;
      SLW   ;
      SPA   I032;
I031: L     DW#16#0;
I032: UD    DW#16#FFFF;
      L     #btPDIData3;
      UD    DW#16#FF;
      OW    ;
      T     #stDataEjector6.wEvacuationTimeT1;
      L     #iStep;
      L     1;
      +I    ;
      T     #iStep;
      SPA   A7d0;
A859: L     44;
      L     LW     2;
      ==I   ;
      SPB   A85b;
      SPA   A85c;
A85b: CLR   ;
      =     DIX [AR2,P#252.6];
      =     DIX [AR2,P#252.7];
      U     DIX [AR2,P#10.5];
      NOT   ;
      SPBN  A7d0;
      L     #iStep;
      L     1;
      +I    ;
      T     #iStep;
      SPA   A7d0;
A85c: L     45;
      L     LW     2;
      ==I   ;
      SPB   A85e;
      SPA   A85f;
A85e: CLR   ;
      =     DIX [AR2,P#252.6];
      SET   ;
      =     DIX [AR2,P#252.7];
      U     DIX [AR2,P#10.5];
      SPBN  A7d0;
      L     #btPDIData2;
      UD    DW#16#FF;
      L     8;
      TAK   ;
      LAR1  ;
      TAK   ;
      L     DW#16#10;
      >=I   ;
      SPB   I033;
      TAK   ;
      TAR1  ;
      SLW   ;
      SPA   I034;
I033: L     DW#16#0;
I034: UD    DW#16#FFFF;
      L     #btPDIData3;
      UD    DW#16#FF;
      OW    ;
      T     #stDataEjector6.wLastFreeFlowVacuum;
      L     #iStep;
      L     1;
      +I    ;
      T     #iStep;
      SPA   A7d0;
A85f: L     46;
      L     LW     2;
      ==I   ;
      SPB   A861;
      SPA   A862;
A861: CLR   ;
      =     DIX [AR2,P#252.6];
      =     DIX [AR2,P#252.7];
      U     DIX [AR2,P#10.5];
      NOT   ;
      SPBN  A7d0;
      L     #iStep;
      L     1;
      +I    ;
      T     #iStep;
      SPA   A7d0;
A862: L     47;
      L     LW     2;
      ==I   ;
      SPB   A864;
      SPA   A865;
A864: SET   ;
      =     DIX [AR2,P#252.6];
      =     DIX [AR2,P#252.7];
      U     DIX [AR2,P#10.5];
      SPBN  A7d0;
      L     #btPDIData1;
      T     #stDataEjector6.btLeakageOfLastCycle;
      L     #btPDIData2;
      UD    DW#16#FF;
      L     8;
      TAK   ;
      LAR1  ;
      TAK   ;
      L     DW#16#10;
      >=I   ;
      SPB   I035;
      TAK   ;
      TAR1  ;
      SLW   ;
      SPA   I036;
I035: L     DW#16#0;
I036: UD    DW#16#FFFF;
      L     #btPDIData3;
      UD    DW#16#FF;
      OW    ;
      T     #stDataEjector6.wAirConsumptionOfLastCyc;
      L     #iStep;
      L     1;
      +I    ;
      T     #iStep;
      SPA   A7d0;
A865: L     48;
      L     LW     2;
      ==I   ;
      SPB   A867;
      SPA   A868;
A867: L     #iNumberOfEjectors;
      L     7;
      >=I   ;
      SPBN  A869;
      L     #iStep;
      L     1;
      +I    ;
      T     #iStep;
      SPA   A7d0;
A869: L     0;
      T     #iStep;
      SPA   A7d0;
A868: L     49;
      L     LW     2;
      ==I   ;
      SPB   A86b;
      SPA   A86c;
A86b: SET   ;
      =     DIX [AR2,P#252.0];
      =     DIX [AR2,P#252.1];
      =     DIX [AR2,P#252.2];
      CLR   ;
      =     DIX [AR2,P#252.3];
      =     DIX [AR2,P#252.4];
      =     DIX [AR2,P#252.6];
      =     DIX [AR2,P#252.7];
      U     DIX [AR2,P#10.5];
      NOT   ;
      SPBN  A7d0;
      L     #btPDIData1;
      T     #stDataEjector7.btErrorByte;
      L     #btPDIData2;
      UD    DW#16#FF;
      L     8;
      TAK   ;
      LAR1  ;
      TAK   ;
      L     DW#16#10;
      >=I   ;
      SPB   I037;
      TAK   ;
      TAR1  ;
      SLW   ;
      SPA   I038;
I037: L     DW#16#0;
I038: UD    DW#16#FFFF;
      L     #btPDIData3;
      UD    DW#16#FF;
      OW    ;
      T     #stDataEjector7.wSystemVacuum;
      L     #iStep;
      L     1;
      +I    ;
      T     #iStep;
      SPA   A7d0;
A86c: L     50;
      L     LW     2;
      ==I   ;
      SPB   A86e;
      SPA   A86f;
A86e: SET   ;
      =     DIX [AR2,P#252.6];
      CLR   ;
      =     DIX [AR2,P#252.7];
      U     DIX [AR2,P#10.5];
      SPBN  A7d0;
      L     #btPDIData1;
      T     #stDataEjector7.btWarningByte;
      L     #btPDIData2;
      UD    DW#16#FF;
      L     8;
      TAK   ;
      LAR1  ;
      TAK   ;
      L     DW#16#10;
      >=I   ;
      SPB   I039;
      TAK   ;
      TAR1  ;
      SLW   ;
      SPA   I03a;
I039: L     DW#16#0;
I03a: UD    DW#16#FFFF;
      L     #btPDIData3;
      UD    DW#16#FF;
      OW    ;
      T     #stDataEjector7.wEvacuationTimeT1;
      L     #iStep;
      L     1;
      +I    ;
      T     #iStep;
      SPA   A7d0;
A86f: L     51;
      L     LW     2;
      ==I   ;
      SPB   A871;
      SPA   A872;
A871: CLR   ;
      =     DIX [AR2,P#252.6];
      =     DIX [AR2,P#252.7];
      U     DIX [AR2,P#10.5];
      NOT   ;
      SPBN  A7d0;
      L     #iStep;
      L     1;
      +I    ;
      T     #iStep;
      SPA   A7d0;
A872: L     52;
      L     LW     2;
      ==I   ;
      SPB   A874;
      SPA   A875;
A874: CLR   ;
      =     DIX [AR2,P#252.6];
      SET   ;
      =     DIX [AR2,P#252.7];
      U     DIX [AR2,P#10.5];
      SPBN  A7d0;
      L     #btPDIData2;
      UD    DW#16#FF;
      L     8;
      TAK   ;
      LAR1  ;
      TAK   ;
      L     DW#16#10;
      >=I   ;
      SPB   I03b;
      TAK   ;
      TAR1  ;
      SLW   ;
      SPA   I03c;
I03b: L     DW#16#0;
I03c: UD    DW#16#FFFF;
      L     #btPDIData3;
      UD    DW#16#FF;
      OW    ;
      T     #stDataEjector7.wLastFreeFlowVacuum;
      L     #iStep;
      L     1;
      +I    ;
      T     #iStep;
      SPA   A7d0;
A875: L     53;
      L     LW     2;
      ==I   ;
      SPB   A877;
      SPA   A878;
A877: CLR   ;
      =     DIX [AR2,P#252.6];
      =     DIX [AR2,P#252.7];
      U     DIX [AR2,P#10.5];
      NOT   ;
      SPBN  A7d0;
      L     #iStep;
      L     1;
      +I    ;
      T     #iStep;
      SPA   A7d0;
A878: L     54;
      L     LW     2;
      ==I   ;
      SPB   A87a;
      SPA   A87b;
A87a: SET   ;
      =     DIX [AR2,P#252.6];
      =     DIX [AR2,P#252.7];
      U     DIX [AR2,P#10.5];
      SPBN  A7d0;
      L     #btPDIData1;
      T     #stDataEjector7.btLeakageOfLastCycle;
      L     #btPDIData2;
      UD    DW#16#FF;
      L     8;
      TAK   ;
      LAR1  ;
      TAK   ;
      L     DW#16#10;
      >=I   ;
      SPB   I03d;
      TAK   ;
      TAR1  ;
      SLW   ;
      SPA   I03e;
I03d: L     DW#16#0;
I03e: UD    DW#16#FFFF;
      L     #btPDIData3;
      UD    DW#16#FF;
      OW    ;
      T     #stDataEjector7.wAirConsumptionOfLastCyc;
      L     #iStep;
      L     1;
      +I    ;
      T     #iStep;
      SPA   A7d0;
A87b: L     55;
      L     LW     2;
      ==I   ;
      SPB   A87d;
      SPA   A87e;
A87d: L     #iNumberOfEjectors;
      L     8;
      >=I   ;
      SPBN  A87f;
      L     #iStep;
      L     1;
      +I    ;
      T     #iStep;
      SPA   A7d0;
A87f: L     0;
      T     #iStep;
      SPA   A7d0;
A87e: L     56;
      L     LW     2;
      ==I   ;
      SPB   A881;
      SPA   A882;
A881: CLR   ;
      =     DIX [AR2,P#252.0];
      =     DIX [AR2,P#252.1];
      =     DIX [AR2,P#252.2];
      SET   ;
      =     DIX [AR2,P#252.3];
      CLR   ;
      =     DIX [AR2,P#252.4];
      =     DIX [AR2,P#252.6];
      =     DIX [AR2,P#252.7];
      U     DIX [AR2,P#10.5];
      NOT   ;
      SPBN  A7d0;
      L     #btPDIData1;
      T     #stDataEjector8.btErrorByte;
      L     #btPDIData2;
      UD    DW#16#FF;
      L     8;
      TAK   ;
      LAR1  ;
      TAK   ;
      L     DW#16#10;
      >=I   ;
      SPB   I03f;
      TAK   ;
      TAR1  ;
      SLW   ;
      SPA   I040;
I03f: L     DW#16#0;
I040: UD    DW#16#FFFF;
      L     #btPDIData3;
      UD    DW#16#FF;
      OW    ;
      T     #stDataEjector8.wSystemVacuum;
      L     #iStep;
      L     1;
      +I    ;
      T     #iStep;
      SPA   A7d0;
A882: L     57;
      L     LW     2;
      ==I   ;
      SPB   A884;
      SPA   A885;
A884: SET   ;
      =     DIX [AR2,P#252.6];
      CLR   ;
      =     DIX [AR2,P#252.7];
      U     DIX [AR2,P#10.5];
      SPBN  A7d0;
      L     #btPDIData1;
      T     #stDataEjector8.btWarningByte;
      L     #btPDIData2;
      UD    DW#16#FF;
      L     8;
      TAK   ;
      LAR1  ;
      TAK   ;
      L     DW#16#10;
      >=I   ;
      SPB   I041;
      TAK   ;
      TAR1  ;
      SLW   ;
      SPA   I042;
I041: L     DW#16#0;
I042: UD    DW#16#FFFF;
      L     #btPDIData3;
      UD    DW#16#FF;
      OW    ;
      T     #stDataEjector8.wEvacuationTimeT1;
      L     #iStep;
      L     1;
      +I    ;
      T     #iStep;
      SPA   A7d0;
A885: L     58;
      L     LW     2;
      ==I   ;
      SPB   A887;
      SPA   A888;
A887: CLR   ;
      =     DIX [AR2,P#252.6];
      =     DIX [AR2,P#252.7];
      U     DIX [AR2,P#10.5];
      NOT   ;
      SPBN  A7d0;
      L     #iStep;
      L     1;
      +I    ;
      T     #iStep;
      SPA   A7d0;
A888: L     59;
      L     LW     2;
      ==I   ;
      SPB   A88a;
      SPA   A88b;
A88a: CLR   ;
      =     DIX [AR2,P#252.6];
      SET   ;
      =     DIX [AR2,P#252.7];
      U     DIX [AR2,P#10.5];
      SPBN  A7d0;
      L     #btPDIData2;
      UD    DW#16#FF;
      L     8;
      TAK   ;
      LAR1  ;
      TAK   ;
      L     DW#16#10;
      >=I   ;
      SPB   I043;
      TAK   ;
      TAR1  ;
      SLW   ;
      SPA   I044;
I043: L     DW#16#0;
I044: UD    DW#16#FFFF;
      L     #btPDIData3;
      UD    DW#16#FF;
      OW    ;
      T     #stDataEjector8.wLastFreeFlowVacuum;
      L     #iStep;
      L     1;
      +I    ;
      T     #iStep;
      SPA   A7d0;
A88b: L     60;
      L     LW     2;
      ==I   ;
      SPB   A88d;
      SPA   A88e;
A88d: CLR   ;
      =     DIX [AR2,P#252.6];
      =     DIX [AR2,P#252.7];
      U     DIX [AR2,P#10.5];
      NOT   ;
      SPBN  A7d0;
      L     #iStep;
      L     1;
      +I    ;
      T     #iStep;
      SPA   A7d0;
A88e: L     61;
      L     LW     2;
      ==I   ;
      SPB   A890;
      SPA   A891;
A890: SET   ;
      =     DIX [AR2,P#252.6];
      =     DIX [AR2,P#252.7];
      U     DIX [AR2,P#10.5];
      SPBN  A7d0;
      L     #btPDIData1;
      T     #stDataEjector8.btLeakageOfLastCycle;
      L     #btPDIData2;
      UD    DW#16#FF;
      L     8;
      TAK   ;
      LAR1  ;
      TAK   ;
      L     DW#16#10;
      >=I   ;
      SPB   I045;
      TAK   ;
      TAR1  ;
      SLW   ;
      SPA   I046;
I045: L     DW#16#0;
I046: UD    DW#16#FFFF;
      L     #btPDIData3;
      UD    DW#16#FF;
      OW    ;
      T     #stDataEjector8.wAirConsumptionOfLastCyc;
      L     #iStep;
      L     1;
      +I    ;
      T     #iStep;
      SPA   A7d0;
A891: L     62;
      L     LW     2;
      ==I   ;
      SPB   A893;
      SPA   A894;
A893: L     #iNumberOfEjectors;
      L     9;
      >=I   ;
      SPBN  A895;
      L     #iStep;
      L     1;
      +I    ;
      T     #iStep;
      SPA   A7d0;
A895: L     0;
      T     #iStep;
      SPA   A7d0;
A894: L     63;
      L     LW     2;
      ==I   ;
      SPB   A897;
      SPA   A898;
A897: SET   ;
      =     DIX [AR2,P#252.0];
      CLR   ;
      =     DIX [AR2,P#252.1];
      =     DIX [AR2,P#252.2];
      SET   ;
      =     DIX [AR2,P#252.3];
      CLR   ;
      =     DIX [AR2,P#252.4];
      =     DIX [AR2,P#252.6];
      =     DIX [AR2,P#252.7];
      U     DIX [AR2,P#10.5];
      NOT   ;
      SPBN  A7d0;
      L     #btPDIData1;
      T     #stDataEjector9.btErrorByte;
      L     #btPDIData2;
      UD    DW#16#FF;
      L     8;
      TAK   ;
      LAR1  ;
      TAK   ;
      L     DW#16#10;
      >=I   ;
      SPB   I047;
      TAK   ;
      TAR1  ;
      SLW   ;
      SPA   I048;
I047: L     DW#16#0;
I048: UD    DW#16#FFFF;
      L     #btPDIData3;
      UD    DW#16#FF;
      OW    ;
      T     #stDataEjector9.wSystemVacuum;
      L     #iStep;
      L     1;
      +I    ;
      T     #iStep;
      SPA   A7d0;
A898: L     64;
      L     LW     2;
      ==I   ;
      SPB   A89a;
      SPA   A89b;
A89a: SET   ;
      =     DIX [AR2,P#252.6];
      CLR   ;
      =     DIX [AR2,P#252.7];
      U     DIX [AR2,P#10.5];
      SPBN  A7d0;
      L     #btPDIData1;
      T     #stDataEjector9.btWarningByte;
      L     #btPDIData2;
      UD    DW#16#FF;
      L     8;
      TAK   ;
      LAR1  ;
      TAK   ;
      L     DW#16#10;
      >=I   ;
      SPB   I049;
      TAK   ;
      TAR1  ;
      SLW   ;
      SPA   I04a;
I049: L     DW#16#0;
I04a: UD    DW#16#FFFF;
      L     #btPDIData3;
      UD    DW#16#FF;
      OW    ;
      T     #stDataEjector9.wEvacuationTimeT1;
      L     #iStep;
      L     1;
      +I    ;
      T     #iStep;
      SPA   A7d0;
A89b: L     65;
      L     LW     2;
      ==I   ;
      SPB   A89d;
      SPA   A89e;
A89d: CLR   ;
      =     DIX [AR2,P#252.6];
      =     DIX [AR2,P#252.7];
      U     DIX [AR2,P#10.5];
      NOT   ;
      SPBN  A7d0;
      L     #iStep;
      L     1;
      +I    ;
      T     #iStep;
      SPA   A7d0;
A89e: L     66;
      L     LW     2;
      ==I   ;
      SPB   A8a0;
      SPA   A8a1;
A8a0: CLR   ;
      =     DIX [AR2,P#252.6];
      SET   ;
      =     DIX [AR2,P#252.7];
      U     DIX [AR2,P#10.5];
      SPBN  A7d0;
      L     #btPDIData2;
      UD    DW#16#FF;
      L     8;
      TAK   ;
      LAR1  ;
      TAK   ;
      L     DW#16#10;
      >=I   ;
      SPB   I04b;
      TAK   ;
      TAR1  ;
      SLW   ;
      SPA   I04c;
I04b: L     DW#16#0;
I04c: UD    DW#16#FFFF;
      L     #btPDIData3;
      UD    DW#16#FF;
      OW    ;
      T     #stDataEjector9.wLastFreeFlowVacuum;
      L     #iStep;
      L     1;
      +I    ;
      T     #iStep;
      SPA   A7d0;
A8a1: L     67;
      L     LW     2;
      ==I   ;
      SPB   A8a3;
      SPA   A8a4;
A8a3: CLR   ;
      =     DIX [AR2,P#252.6];
      =     DIX [AR2,P#252.7];
      U     DIX [AR2,P#10.5];
      NOT   ;
      SPBN  A7d0;
      L     #iStep;
      L     1;
      +I    ;
      T     #iStep;
      SPA   A7d0;
A8a4: L     68;
      L     LW     2;
      ==I   ;
      SPB   A8a6;
      SPA   A8a7;
A8a6: SET   ;
      =     DIX [AR2,P#252.6];
      =     DIX [AR2,P#252.7];
      U     DIX [AR2,P#10.5];
      SPBN  A7d0;
      L     #btPDIData1;
      T     #stDataEjector9.btLeakageOfLastCycle;
      L     #btPDIData2;
      UD    DW#16#FF;
      L     8;
      TAK   ;
      LAR1  ;
      TAK   ;
      L     DW#16#10;
      >=I   ;
      SPB   I04d;
      TAK   ;
      TAR1  ;
      SLW   ;
      SPA   I04e;
I04d: L     DW#16#0;
I04e: UD    DW#16#FFFF;
      L     #btPDIData3;
      UD    DW#16#FF;
      OW    ;
      T     #stDataEjector9.wAirConsumptionOfLastCyc;
      L     #iStep;
      L     1;
      +I    ;
      T     #iStep;
      SPA   A7d0;
A8a7: L     69;
      L     LW     2;
      ==I   ;
      SPB   A8a9;
      SPA   A8aa;
A8a9: L     #iNumberOfEjectors;
      L     10;
      >=I   ;
      SPBN  A8ab;
      L     #iStep;
      L     1;
      +I    ;
      T     #iStep;
      SPA   A7d0;
A8ab: L     0;
      T     #iStep;
      SPA   A7d0;
A8aa: L     70;
      L     LW     2;
      ==I   ;
      SPB   A8ad;
      SPA   A8ae;
A8ad: CLR   ;
      =     DIX [AR2,P#252.0];
      SET   ;
      =     DIX [AR2,P#252.1];
      CLR   ;
      =     DIX [AR2,P#252.2];
      SET   ;
      =     DIX [AR2,P#252.3];
      CLR   ;
      =     DIX [AR2,P#252.4];
      =     DIX [AR2,P#252.6];
      =     DIX [AR2,P#252.7];
      U     DIX [AR2,P#10.5];
      NOT   ;
      SPBN  A7d0;
      L     #btPDIData1;
      T     #stDataEjector10.btErrorByte;
      L     #btPDIData2;
      UD    DW#16#FF;
      L     8;
      TAK   ;
      LAR1  ;
      TAK   ;
      L     DW#16#10;
      >=I   ;
      SPB   I04f;
      TAK   ;
      TAR1  ;
      SLW   ;
      SPA   I050;
I04f: L     DW#16#0;
I050: UD    DW#16#FFFF;
      L     #btPDIData3;
      UD    DW#16#FF;
      OW    ;
      T     #stDataEjector10.wSystemVacuum;
      L     #iStep;
      L     1;
      +I    ;
      T     #iStep;
      SPA   A7d0;
A8ae: L     71;
      L     LW     2;
      ==I   ;
      SPB   A8b0;
      SPA   A8b1;
A8b0: SET   ;
      =     DIX [AR2,P#252.6];
      CLR   ;
      =     DIX [AR2,P#252.7];
      U     DIX [AR2,P#10.5];
      SPBN  A7d0;
      L     #btPDIData1;
      T     #stDataEjector10.btWarningByte;
      L     #btPDIData2;
      UD    DW#16#FF;
      L     8;
      TAK   ;
      LAR1  ;
      TAK   ;
      L     DW#16#10;
      >=I   ;
      SPB   I051;
      TAK   ;
      TAR1  ;
      SLW   ;
      SPA   I052;
I051: L     DW#16#0;
I052: UD    DW#16#FFFF;
      L     #btPDIData3;
      UD    DW#16#FF;
      OW    ;
      T     #stDataEjector10.wEvacuationTimeT1;
      L     #iStep;
      L     1;
      +I    ;
      T     #iStep;
      SPA   A7d0;
A8b1: L     72;
      L     LW     2;
      ==I   ;
      SPB   A8b3;
      SPA   A8b4;
A8b3: CLR   ;
      =     DIX [AR2,P#252.6];
      =     DIX [AR2,P#252.7];
      U     DIX [AR2,P#10.5];
      NOT   ;
      SPBN  A7d0;
      L     #iStep;
      L     1;
      +I    ;
      T     #iStep;
      SPA   A7d0;
A8b4: L     73;
      L     LW     2;
      ==I   ;
      SPB   A8b6;
      SPA   A8b7;
A8b6: CLR   ;
      =     DIX [AR2,P#252.6];
      SET   ;
      =     DIX [AR2,P#252.7];
      U     DIX [AR2,P#10.5];
      SPBN  A7d0;
      L     #btPDIData2;
      UD    DW#16#FF;
      L     8;
      TAK   ;
      LAR1  ;
      TAK   ;
      L     DW#16#10;
      >=I   ;
      SPB   I053;
      TAK   ;
      TAR1  ;
      SLW   ;
      SPA   I054;
I053: L     DW#16#0;
I054: UD    DW#16#FFFF;
      L     #btPDIData3;
      UD    DW#16#FF;
      OW    ;
      T     #stDataEjector10.wLastFreeFlowVacuum;
      L     #iStep;
      L     1;
      +I    ;
      T     #iStep;
      SPA   A7d0;
A8b7: L     74;
      L     LW     2;
      ==I   ;
      SPB   A8b9;
      SPA   A8ba;
A8b9: CLR   ;
      =     DIX [AR2,P#252.6];
      =     DIX [AR2,P#252.7];
      U     DIX [AR2,P#10.5];
      NOT   ;
      SPBN  A7d0;
      L     #iStep;
      L     1;
      +I    ;
      T     #iStep;
      SPA   A7d0;
A8ba: L     75;
      L     LW     2;
      ==I   ;
      SPB   A8bc;
      SPA   A8bd;
A8bc: SET   ;
      =     DIX [AR2,P#252.6];
      =     DIX [AR2,P#252.7];
      U     DIX [AR2,P#10.5];
      SPBN  A7d0;
      L     #btPDIData1;
      T     #stDataEjector10.btLeakageOfLastCycle;
      L     #btPDIData2;
      UD    DW#16#FF;
      L     8;
      TAK   ;
      LAR1  ;
      TAK   ;
      L     DW#16#10;
      >=I   ;
      SPB   I055;
      TAK   ;
      TAR1  ;
      SLW   ;
      SPA   I056;
I055: L     DW#16#0;
I056: UD    DW#16#FFFF;
      L     #btPDIData3;
      UD    DW#16#FF;
      OW    ;
      T     #stDataEjector10.wAirConsumptionOfLastCyc;
      L     #iStep;
      L     1;
      +I    ;
      T     #iStep;
      SPA   A7d0;
A8bd: L     76;
      L     LW     2;
      ==I   ;
      SPB   A8bf;
      SPA   A8c0;
A8bf: L     #iNumberOfEjectors;
      L     11;
      >=I   ;
      SPBN  A8c1;
      L     #iStep;
      L     1;
      +I    ;
      T     #iStep;
      SPA   A7d0;
A8c1: L     0;
      T     #iStep;
      SPA   A7d0;
A8c0: L     77;
      L     LW     2;
      ==I   ;
      SPB   A8c3;
      SPA   A8c4;
A8c3: SET   ;
      =     DIX [AR2,P#252.0];
      =     DIX [AR2,P#252.1];
      CLR   ;
      =     DIX [AR2,P#252.2];
      SET   ;
      =     DIX [AR2,P#252.3];
      CLR   ;
      =     DIX [AR2,P#252.4];
      =     DIX [AR2,P#252.6];
      =     DIX [AR2,P#252.7];
      U     DIX [AR2,P#10.5];
      NOT   ;
      SPBN  A7d0;
      L     #btPDIData1;
      T     #stDataEjector11.btErrorByte;
      L     #btPDIData2;
      UD    DW#16#FF;
      L     8;
      TAK   ;
      LAR1  ;
      TAK   ;
      L     DW#16#10;
      >=I   ;
      SPB   I057;
      TAK   ;
      TAR1  ;
      SLW   ;
      SPA   I058;
I057: L     DW#16#0;
I058: UD    DW#16#FFFF;
      L     #btPDIData3;
      UD    DW#16#FF;
      OW    ;
      T     #stDataEjector11.wSystemVacuum;
      L     #iStep;
      L     1;
      +I    ;
      T     #iStep;
      SPA   A7d0;
A8c4: L     78;
      L     LW     2;
      ==I   ;
      SPB   A8c6;
      SPA   A8c7;
A8c6: SET   ;
      =     DIX [AR2,P#252.6];
      CLR   ;
      =     DIX [AR2,P#252.7];
      U     DIX [AR2,P#10.5];
      SPBN  A7d0;
      L     #btPDIData1;
      T     #stDataEjector11.btWarningByte;
      L     #btPDIData2;
      UD    DW#16#FF;
      L     8;
      TAK   ;
      LAR1  ;
      TAK   ;
      L     DW#16#10;
      >=I   ;
      SPB   I059;
      TAK   ;
      TAR1  ;
      SLW   ;
      SPA   I05a;
I059: L     DW#16#0;
I05a: UD    DW#16#FFFF;
      L     #btPDIData3;
      UD    DW#16#FF;
      OW    ;
      T     #stDataEjector11.wEvacuationTimeT1;
      L     #iStep;
      L     1;
      +I    ;
      T     #iStep;
      SPA   A7d0;
A8c7: L     79;
      L     LW     2;
      ==I   ;
      SPB   A8c9;
      SPA   A8ca;
A8c9: CLR   ;
      =     DIX [AR2,P#252.6];
      =     DIX [AR2,P#252.7];
      U     DIX [AR2,P#10.5];
      NOT   ;
      SPBN  A7d0;
      L     #iStep;
      L     1;
      +I    ;
      T     #iStep;
      SPA   A7d0;
A8ca: L     80;
      L     LW     2;
      ==I   ;
      SPB   A8cc;
      SPA   A8cd;
A8cc: CLR   ;
      =     DIX [AR2,P#252.6];
      SET   ;
      =     DIX [AR2,P#252.7];
      U     DIX [AR2,P#10.5];
      SPBN  A7d0;
      L     #btPDIData2;
      UD    DW#16#FF;
      L     8;
      TAK   ;
      LAR1  ;
      TAK   ;
      L     DW#16#10;
      >=I   ;
      SPB   I05b;
      TAK   ;
      TAR1  ;
      SLW   ;
      SPA   I05c;
I05b: L     DW#16#0;
I05c: UD    DW#16#FFFF;
      L     #btPDIData3;
      UD    DW#16#FF;
      OW    ;
      T     #stDataEjector11.wLastFreeFlowVacuum;
      L     #iStep;
      L     1;
      +I    ;
      T     #iStep;
      SPA   A7d0;
A8cd: L     81;
      L     LW     2;
      ==I   ;
      SPB   A8cf;
      SPA   A8d0;
A8cf: CLR   ;
      =     DIX [AR2,P#252.6];
      =     DIX [AR2,P#252.7];
      U     DIX [AR2,P#10.5];
      NOT   ;
      SPBN  A7d0;
      L     #iStep;
      L     1;
      +I    ;
      T     #iStep;
      SPA   A7d0;
A8d0: L     82;
      L     LW     2;
      ==I   ;
      SPB   A8d2;
      SPA   A8d3;
A8d2: SET   ;
      =     DIX [AR2,P#252.6];
      =     DIX [AR2,P#252.7];
      U     DIX [AR2,P#10.5];
      SPBN  A7d0;
      L     #btPDIData1;
      T     #stDataEjector11.btLeakageOfLastCycle;
      L     #btPDIData2;
      UD    DW#16#FF;
      L     8;
      TAK   ;
      LAR1  ;
      TAK   ;
      L     DW#16#10;
      >=I   ;
      SPB   I05d;
      TAK   ;
      TAR1  ;
      SLW   ;
      SPA   I05e;
I05d: L     DW#16#0;
I05e: UD    DW#16#FFFF;
      L     #btPDIData3;
      UD    DW#16#FF;
      OW    ;
      T     #stDataEjector11.wAirConsumptionOfLastCyc;
      L     #iStep;
      L     1;
      +I    ;
      T     #iStep;
      SPA   A7d0;
A8d3: L     83;
      L     LW     2;
      ==I   ;
      SPB   A8d5;
      SPA   A8d6;
A8d5: L     #iNumberOfEjectors;
      L     12;
      >=I   ;
      SPBN  A8d7;
      L     #iStep;
      L     1;
      +I    ;
      T     #iStep;
      SPA   A7d0;
A8d7: L     0;
      T     #iStep;
      SPA   A7d0;
A8d6: L     84;
      L     LW     2;
      ==I   ;
      SPB   A8d9;
      SPA   A8da;
A8d9: CLR   ;
      =     DIX [AR2,P#252.0];
      =     DIX [AR2,P#252.1];
      SET   ;
      =     DIX [AR2,P#252.2];
      =     DIX [AR2,P#252.3];
      CLR   ;
      =     DIX [AR2,P#252.4];
      =     DIX [AR2,P#252.6];
      =     DIX [AR2,P#252.7];
      U     DIX [AR2,P#10.5];
      NOT   ;
      SPBN  A7d0;
      L     #btPDIData1;
      T     #stDataEjector12.btErrorByte;
      L     #btPDIData2;
      UD    DW#16#FF;
      L     8;
      TAK   ;
      LAR1  ;
      TAK   ;
      L     DW#16#10;
      >=I   ;
      SPB   I05f;
      TAK   ;
      TAR1  ;
      SLW   ;
      SPA   I060;
I05f: L     DW#16#0;
I060: UD    DW#16#FFFF;
      L     #btPDIData3;
      UD    DW#16#FF;
      OW    ;
      T     #stDataEjector12.wSystemVacuum;
      L     #iStep;
      L     1;
      +I    ;
      T     #iStep;
      SPA   A7d0;
A8da: L     85;
      L     LW     2;
      ==I   ;
      SPB   A8dc;
      SPA   A8dd;
A8dc: SET   ;
      =     DIX [AR2,P#252.6];
      CLR   ;
      =     DIX [AR2,P#252.7];
      U     DIX [AR2,P#10.5];
      SPBN  A7d0;
      L     #btPDIData1;
      T     #stDataEjector12.btWarningByte;
      L     #btPDIData2;
      UD    DW#16#FF;
      L     8;
      TAK   ;
      LAR1  ;
      TAK   ;
      L     DW#16#10;
      >=I   ;
      SPB   I061;
      TAK   ;
      TAR1  ;
      SLW   ;
      SPA   I062;
I061: L     DW#16#0;
I062: UD    DW#16#FFFF;
      L     #btPDIData3;
      UD    DW#16#FF;
      OW    ;
      T     #stDataEjector12.wEvacuationTimeT1;
      L     #iStep;
      L     1;
      +I    ;
      T     #iStep;
      SPA   A7d0;
A8dd: L     86;
      L     LW     2;
      ==I   ;
      SPB   A8df;
      SPA   A8e0;
A8df: CLR   ;
      =     DIX [AR2,P#252.6];
      =     DIX [AR2,P#252.7];
      U     DIX [AR2,P#10.5];
      NOT   ;
      SPBN  A7d0;
      L     #iStep;
      L     1;
      +I    ;
      T     #iStep;
      SPA   A7d0;
A8e0: L     87;
      L     LW     2;
      ==I   ;
      SPB   A8e2;
      SPA   A8e3;
A8e2: CLR   ;
      =     DIX [AR2,P#252.6];
      SET   ;
      =     DIX [AR2,P#252.7];
      U     DIX [AR2,P#10.5];
      SPBN  A7d0;
      L     #btPDIData2;
      UD    DW#16#FF;
      L     8;
      TAK   ;
      LAR1  ;
      TAK   ;
      L     DW#16#10;
      >=I   ;
      SPB   I063;
      TAK   ;
      TAR1  ;
      SLW   ;
      SPA   I064;
I063: L     DW#16#0;
I064: UD    DW#16#FFFF;
      L     #btPDIData3;
      UD    DW#16#FF;
      OW    ;
      T     #stDataEjector12.wLastFreeFlowVacuum;
      L     #iStep;
      L     1;
      +I    ;
      T     #iStep;
      SPA   A7d0;
A8e3: L     88;
      L     LW     2;
      ==I   ;
      SPB   A8e5;
      SPA   A8e6;
A8e5: CLR   ;
      =     DIX [AR2,P#252.6];
      =     DIX [AR2,P#252.7];
      U     DIX [AR2,P#10.5];
      NOT   ;
      SPBN  A7d0;
      L     #iStep;
      L     1;
      +I    ;
      T     #iStep;
      SPA   A7d0;
A8e6: L     89;
      L     LW     2;
      ==I   ;
      SPB   A8e8;
      SPA   A8e9;
A8e8: SET   ;
      =     DIX [AR2,P#252.6];
      =     DIX [AR2,P#252.7];
      U     DIX [AR2,P#10.5];
      SPBN  A7d0;
      L     #btPDIData1;
      T     #stDataEjector12.btLeakageOfLastCycle;
      L     #btPDIData2;
      UD    DW#16#FF;
      L     8;
      TAK   ;
      LAR1  ;
      TAK   ;
      L     DW#16#10;
      >=I   ;
      SPB   I065;
      TAK   ;
      TAR1  ;
      SLW   ;
      SPA   I066;
I065: L     DW#16#0;
I066: UD    DW#16#FFFF;
      L     #btPDIData3;
      UD    DW#16#FF;
      OW    ;
      T     #stDataEjector12.wAirConsumptionOfLastCyc;
      L     #iStep;
      L     1;
      +I    ;
      T     #iStep;
      SPA   A7d0;
A8e9: L     90;
      L     LW     2;
      ==I   ;
      SPB   A8eb;
      SPA   A8ec;
A8eb: L     #iNumberOfEjectors;
      L     13;
      >=I   ;
      SPBN  A8ed;
      L     #iStep;
      L     1;
      +I    ;
      T     #iStep;
      SPA   A7d0;
A8ed: L     0;
      T     #iStep;
      SPA   A7d0;
A8ec: L     91;
      L     LW     2;
      ==I   ;
      SPB   A8ef;
      SPA   A8f0;
A8ef: SET   ;
      =     DIX [AR2,P#252.0];
      CLR   ;
      =     DIX [AR2,P#252.1];
      SET   ;
      =     DIX [AR2,P#252.2];
      =     DIX [AR2,P#252.3];
      CLR   ;
      =     DIX [AR2,P#252.4];
      =     DIX [AR2,P#252.6];
      =     DIX [AR2,P#252.7];
      U     DIX [AR2,P#10.5];
      NOT   ;
      SPBN  A7d0;
      L     #btPDIData1;
      T     #stDataEjector13.btErrorByte;
      L     #btPDIData2;
      UD    DW#16#FF;
      L     8;
      TAK   ;
      LAR1  ;
      TAK   ;
      L     DW#16#10;
      >=I   ;
      SPB   I067;
      TAK   ;
      TAR1  ;
      SLW   ;
      SPA   I068;
I067: L     DW#16#0;
I068: UD    DW#16#FFFF;
      L     #btPDIData3;
      UD    DW#16#FF;
      OW    ;
      T     #stDataEjector13.wSystemVacuum;
      L     #iStep;
      L     1;
      +I    ;
      T     #iStep;
      SPA   A7d0;
A8f0: L     92;
      L     LW     2;
      ==I   ;
      SPB   A8f2;
      SPA   A8f3;
A8f2: SET   ;
      =     DIX [AR2,P#252.6];
      CLR   ;
      =     DIX [AR2,P#252.7];
      U     DIX [AR2,P#10.5];
      SPBN  A7d0;
      L     #btPDIData1;
      T     #stDataEjector13.btWarningByte;
      L     #btPDIData2;
      UD    DW#16#FF;
      L     8;
      TAK   ;
      LAR1  ;
      TAK   ;
      L     DW#16#10;
      >=I   ;
      SPB   I069;
      TAK   ;
      TAR1  ;
      SLW   ;
      SPA   I06a;
I069: L     DW#16#0;
I06a: UD    DW#16#FFFF;
      L     #btPDIData3;
      UD    DW#16#FF;
      OW    ;
      T     #stDataEjector13.wEvacuationTimeT1;
      L     #iStep;
      L     1;
      +I    ;
      T     #iStep;
      SPA   A7d0;
A8f3: L     93;
      L     LW     2;
      ==I   ;
      SPB   A8f5;
      SPA   A8f6;
A8f5: CLR   ;
      =     DIX [AR2,P#252.6];
      =     DIX [AR2,P#252.7];
      U     DIX [AR2,P#10.5];
      NOT   ;
      SPBN  A7d0;
      L     #iStep;
      L     1;
      +I    ;
      T     #iStep;
      SPA   A7d0;
A8f6: L     94;
      L     LW     2;
      ==I   ;
      SPB   A8f8;
      SPA   A8f9;
A8f8: CLR   ;
      =     DIX [AR2,P#252.6];
      SET   ;
      =     DIX [AR2,P#252.7];
      U     DIX [AR2,P#10.5];
      SPBN  A7d0;
      L     #btPDIData2;
      UD    DW#16#FF;
      L     8;
      TAK   ;
      LAR1  ;
      TAK   ;
      L     DW#16#10;
      >=I   ;
      SPB   I06b;
      TAK   ;
      TAR1  ;
      SLW   ;
      SPA   I06c;
I06b: L     DW#16#0;
I06c: UD    DW#16#FFFF;
      L     #btPDIData3;
      UD    DW#16#FF;
      OW    ;
      T     #stDataEjector13.wLastFreeFlowVacuum;
      L     #iStep;
      L     1;
      +I    ;
      T     #iStep;
      SPA   A7d0;
A8f9: L     95;
      L     LW     2;
      ==I   ;
      SPB   A8fb;
      SPA   A8fc;
A8fb: CLR   ;
      =     DIX [AR2,P#252.6];
      =     DIX [AR2,P#252.7];
      U     DIX [AR2,P#10.5];
      NOT   ;
      SPBN  A7d0;
      L     #iStep;
      L     1;
      +I    ;
      T     #iStep;
      SPA   A7d0;
A8fc: L     96;
      L     LW     2;
      ==I   ;
      SPB   A8fe;
      SPA   A8ff;
A8fe: SET   ;
      =     DIX [AR2,P#252.6];
      =     DIX [AR2,P#252.7];
      U     DIX [AR2,P#10.5];
      SPBN  A7d0;
      L     #btPDIData1;
      T     #stDataEjector13.btLeakageOfLastCycle;
      L     #btPDIData2;
      UD    DW#16#FF;
      L     8;
      TAK   ;
      LAR1  ;
      TAK   ;
      L     DW#16#10;
      >=I   ;
      SPB   I06d;
      TAK   ;
      TAR1  ;
      SLW   ;
      SPA   I06e;
I06d: L     DW#16#0;
I06e: UD    DW#16#FFFF;
      L     #btPDIData3;
      UD    DW#16#FF;
      OW    ;
      T     #stDataEjector13.wAirConsumptionOfLastCyc;
      L     #iStep;
      L     1;
      +I    ;
      T     #iStep;
      SPA   A7d0;
A8ff: L     97;
      L     LW     2;
      ==I   ;
      SPB   A901;
      SPA   A902;
A901: L     #iNumberOfEjectors;
      L     14;
      >=I   ;
      SPBN  A903;
      L     #iStep;
      L     1;
      +I    ;
      T     #iStep;
      SPA   A7d0;
A903: L     0;
      T     #iStep;
      SPA   A7d0;
A902: L     98;
      L     LW     2;
      ==I   ;
      SPB   A905;
      SPA   A906;
A905: CLR   ;
      =     DIX [AR2,P#252.0];
      SET   ;
      =     DIX [AR2,P#252.1];
      =     DIX [AR2,P#252.2];
      =     DIX [AR2,P#252.3];
      CLR   ;
      =     DIX [AR2,P#252.4];
      =     DIX [AR2,P#252.6];
      =     DIX [AR2,P#252.7];
      U     DIX [AR2,P#10.5];
      NOT   ;
      SPBN  A7d0;
      L     #btPDIData1;
      T     #stDataEjector14.btErrorByte;
      L     #btPDIData2;
      UD    DW#16#FF;
      L     8;
      TAK   ;
      LAR1  ;
      TAK   ;
      L     DW#16#10;
      >=I   ;
      SPB   I06f;
      TAK   ;
      TAR1  ;
      SLW   ;
      SPA   I070;
I06f: L     DW#16#0;
I070: UD    DW#16#FFFF;
      L     #btPDIData3;
      UD    DW#16#FF;
      OW    ;
      T     #stDataEjector14.wSystemVacuum;
      L     #iStep;
      L     1;
      +I    ;
      T     #iStep;
      SPA   A7d0;
A906: L     99;
      L     LW     2;
      ==I   ;
      SPB   A908;
      SPA   A909;
A908: SET   ;
      =     DIX [AR2,P#252.6];
      CLR   ;
      =     DIX [AR2,P#252.7];
      U     DIX [AR2,P#10.5];
      SPBN  A7d0;
      L     #btPDIData1;
      T     #stDataEjector14.btWarningByte;
      L     #btPDIData2;
      UD    DW#16#FF;
      L     8;
      TAK   ;
      LAR1  ;
      TAK   ;
      L     DW#16#10;
      >=I   ;
      SPB   I071;
      TAK   ;
      TAR1  ;
      SLW   ;
      SPA   I072;
I071: L     DW#16#0;
I072: UD    DW#16#FFFF;
      L     #btPDIData3;
      UD    DW#16#FF;
      OW    ;
      T     #stDataEjector14.wEvacuationTimeT1;
      L     #iStep;
      L     1;
      +I    ;
      T     #iStep;
      SPA   A7d0;
A909: L     100;
      L     LW     2;
      ==I   ;
      SPB   A90b;
      SPA   A90c;
A90b: CLR   ;
      =     DIX [AR2,P#252.6];
      =     DIX [AR2,P#252.7];
      U     DIX [AR2,P#10.5];
      NOT   ;
      SPBN  A7d0;
      L     #iStep;
      L     1;
      +I    ;
      T     #iStep;
      SPA   A7d0;
A90c: L     101;
      L     LW     2;
      ==I   ;
      SPB   A90e;
      SPA   A90f;
A90e: CLR   ;
      =     DIX [AR2,P#252.6];
      SET   ;
      =     DIX [AR2,P#252.7];
      U     DIX [AR2,P#10.5];
      SPBN  A7d0;
      L     #btPDIData2;
      UD    DW#16#FF;
      L     8;
      TAK   ;
      LAR1  ;
      TAK   ;
      L     DW#16#10;
      >=I   ;
      SPB   I073;
      TAK   ;
      TAR1  ;
      SLW   ;
      SPA   I074;
I073: L     DW#16#0;
I074: UD    DW#16#FFFF;
      L     #btPDIData3;
      UD    DW#16#FF;
      OW    ;
      T     #stDataEjector14.wLastFreeFlowVacuum;
      L     #iStep;
      L     1;
      +I    ;
      T     #iStep;
      SPA   A7d0;
A90f: L     102;
      L     LW     2;
      ==I   ;
      SPB   A911;
      SPA   A912;
A911: CLR   ;
      =     DIX [AR2,P#252.6];
      =     DIX [AR2,P#252.7];
      U     DIX [AR2,P#10.5];
      NOT   ;
      SPBN  A7d0;
      L     #iStep;
      L     1;
      +I    ;
      T     #iStep;
      SPA   A7d0;
A912: L     103;
      L     LW     2;
      ==I   ;
      SPB   A914;
      SPA   A915;
A914: SET   ;
      =     DIX [AR2,P#252.6];
      =     DIX [AR2,P#252.7];
      U     DIX [AR2,P#10.5];
      SPBN  A7d0;
      L     #btPDIData1;
      T     #stDataEjector14.btLeakageOfLastCycle;
      L     #btPDIData2;
      UD    DW#16#FF;
      L     8;
      TAK   ;
      LAR1  ;
      TAK   ;
      L     DW#16#10;
      >=I   ;
      SPB   I075;
      TAK   ;
      TAR1  ;
      SLW   ;
      SPA   I076;
I075: L     DW#16#0;
I076: UD    DW#16#FFFF;
      L     #btPDIData3;
      UD    DW#16#FF;
      OW    ;
      T     #stDataEjector14.wAirConsumptionOfLastCyc;
      L     #iStep;
      L     1;
      +I    ;
      T     #iStep;
      SPA   A7d0;
A915: L     104;
      L     LW     2;
      ==I   ;
      SPB   A917;
      SPA   A918;
A917: L     #iNumberOfEjectors;
      L     15;
      >=I   ;
      SPBN  A919;
      L     #iStep;
      L     1;
      +I    ;
      T     #iStep;
      SPA   A7d0;
A919: L     0;
      T     #iStep;
      SPA   A7d0;
A918: L     105;
      L     LW     2;
      ==I   ;
      SPB   A91b;
      SPA   A91c;
A91b: SET   ;
      =     DIX [AR2,P#252.0];
      =     DIX [AR2,P#252.1];
      =     DIX [AR2,P#252.2];
      =     DIX [AR2,P#252.3];
      CLR   ;
      =     DIX [AR2,P#252.4];
      =     DIX [AR2,P#252.6];
      =     DIX [AR2,P#252.7];
      U     DIX [AR2,P#10.5];
      NOT   ;
      SPBN  A7d0;
      L     #btPDIData1;
      T     #stDataEjector15.btErrorByte;
      L     #btPDIData2;
      UD    DW#16#FF;
      L     8;
      TAK   ;
      LAR1  ;
      TAK   ;
      L     DW#16#10;
      >=I   ;
      SPB   I077;
      TAK   ;
      TAR1  ;
      SLW   ;
      SPA   I078;
I077: L     DW#16#0;
I078: UD    DW#16#FFFF;
      L     #btPDIData3;
      UD    DW#16#FF;
      OW    ;
      T     #stDataEjector15.wSystemVacuum;
      L     #iStep;
      L     1;
      +I    ;
      T     #iStep;
      SPA   A7d0;
A91c: L     106;
      L     LW     2;
      ==I   ;
      SPB   A91e;
      SPA   A91f;
A91e: SET   ;
      =     DIX [AR2,P#252.6];
      CLR   ;
      =     DIX [AR2,P#252.7];
      U     DIX [AR2,P#10.5];
      SPBN  A7d0;
      L     #btPDIData1;
      T     #stDataEjector15.btWarningByte;
      L     #btPDIData2;
      UD    DW#16#FF;
      L     8;
      TAK   ;
      LAR1  ;
      TAK   ;
      L     DW#16#10;
      >=I   ;
      SPB   I079;
      TAK   ;
      TAR1  ;
      SLW   ;
      SPA   I07a;
I079: L     DW#16#0;
I07a: UD    DW#16#FFFF;
      L     #btPDIData3;
      UD    DW#16#FF;
      OW    ;
      T     #stDataEjector15.wEvacuationTimeT1;
      L     #iStep;
      L     1;
      +I    ;
      T     #iStep;
      SPA   A7d0;
A91f: L     107;
      L     LW     2;
      ==I   ;
      SPB   A921;
      SPA   A922;
A921: CLR   ;
      =     DIX [AR2,P#252.6];
      =     DIX [AR2,P#252.7];
      U     DIX [AR2,P#10.5];
      NOT   ;
      SPBN  A7d0;
      L     #iStep;
      L     1;
      +I    ;
      T     #iStep;
      SPA   A7d0;
A922: L     108;
      L     LW     2;
      ==I   ;
      SPB   A924;
      SPA   A925;
A924: CLR   ;
      =     DIX [AR2,P#252.6];
      SET   ;
      =     DIX [AR2,P#252.7];
      U     DIX [AR2,P#10.5];
      SPBN  A7d0;
      L     #btPDIData2;
      UD    DW#16#FF;
      L     8;
      TAK   ;
      LAR1  ;
      TAK   ;
      L     DW#16#10;
      >=I   ;
      SPB   I07b;
      TAK   ;
      TAR1  ;
      SLW   ;
      SPA   I07c;
I07b: L     DW#16#0;
I07c: UD    DW#16#FFFF;
      L     #btPDIData3;
      UD    DW#16#FF;
      OW    ;
      T     #stDataEjector15.wLastFreeFlowVacuum;
      L     #iStep;
      L     1;
      +I    ;
      T     #iStep;
      SPA   A7d0;
A925: L     109;
      L     LW     2;
      ==I   ;
      SPB   A927;
      SPA   A928;
A927: CLR   ;
      =     DIX [AR2,P#252.6];
      =     DIX [AR2,P#252.7];
      U     DIX [AR2,P#10.5];
      NOT   ;
      SPBN  A7d0;
      L     #iStep;
      L     1;
      +I    ;
      T     #iStep;
      SPA   A7d0;
A928: L     110;
      L     LW     2;
      ==I   ;
      SPB   A92a;
      SPA   A92b;
A92a: SET   ;
      =     DIX [AR2,P#252.6];
      =     DIX [AR2,P#252.7];
      U     DIX [AR2,P#10.5];
      SPBN  A7d0;
      L     #btPDIData1;
      T     #stDataEjector15.btLeakageOfLastCycle;
      L     #btPDIData2;
      UD    DW#16#FF;
      L     8;
      TAK   ;
      LAR1  ;
      TAK   ;
      L     DW#16#10;
      >=I   ;
      SPB   I07d;
      TAK   ;
      TAR1  ;
      SLW   ;
      SPA   I07e;
I07d: L     DW#16#0;
I07e: UD    DW#16#FFFF;
      L     #btPDIData3;
      UD    DW#16#FF;
      OW    ;
      T     #stDataEjector15.wAirConsumptionOfLastCyc;
      L     #iStep;
      L     1;
      +I    ;
      T     #iStep;
      SPA   A7d0;
A92b: L     111;
      L     LW     2;
      ==I   ;
      SPB   A92d;
      SPA   A92e;
A92d: L     #iNumberOfEjectors;
      L     16;
      ==I   ;
      SPBN  A92f;
      L     #iStep;
      L     1;
      +I    ;
      T     #iStep;
      SPA   A7d0;
A92f: L     0;
      T     #iStep;
      SPA   A7d0;
A92e: L     112;
      L     LW     2;
      ==I   ;
      SPB   A931;
      SPA   A932;
A931: CLR   ;
      =     DIX [AR2,P#252.0];
      =     DIX [AR2,P#252.1];
      =     DIX [AR2,P#252.2];
      =     DIX [AR2,P#252.3];
      SET   ;
      =     DIX [AR2,P#252.4];
      CLR   ;
      =     DIX [AR2,P#252.6];
      =     DIX [AR2,P#252.7];
      U     DIX [AR2,P#10.5];
      NOT   ;
      SPBN  A7d0;
      L     #btPDIData1;
      T     #stDataEjector16.btErrorByte;
      L     #btPDIData2;
      UD    DW#16#FF;
      L     8;
      TAK   ;
      LAR1  ;
      TAK   ;
      L     DW#16#10;
      >=I   ;
      SPB   I07f;
      TAK   ;
      TAR1  ;
      SLW   ;
      SPA   I080;
I07f: L     DW#16#0;
I080: UD    DW#16#FFFF;
      L     #btPDIData3;
      UD    DW#16#FF;
      OW    ;
      T     #stDataEjector16.wSystemVacuum;
      L     #iStep;
      L     1;
      +I    ;
      T     #iStep;
      SPA   A7d0;
A932: L     113;
      L     LW     2;
      ==I   ;
      SPB   A934;
      SPA   A935;
A934: SET   ;
      =     DIX [AR2,P#252.6];
      CLR   ;
      =     DIX [AR2,P#252.7];
      U     DIX [AR2,P#10.5];
      SPBN  A7d0;
      L     #btPDIData1;
      T     #stDataEjector16.btWarningByte;
      L     #btPDIData2;
      UD    DW#16#FF;
      L     8;
      TAK   ;
      LAR1  ;
      TAK   ;
      L     DW#16#10;
      >=I   ;
      SPB   I081;
      TAK   ;
      TAR1  ;
      SLW   ;
      SPA   I082;
I081: L     DW#16#0;
I082: UD    DW#16#FFFF;
      L     #btPDIData3;
      UD    DW#16#FF;
      OW    ;
      T     #stDataEjector16.wEvacuationTimeT1;
      L     #iStep;
      L     1;
      +I    ;
      T     #iStep;
      SPA   A7d0;
A935: L     114;
      L     LW     2;
      ==I   ;
      SPB   A937;
      SPA   A938;
A937: CLR   ;
      =     DIX [AR2,P#252.6];
      =     DIX [AR2,P#252.7];
      U     DIX [AR2,P#10.5];
      NOT   ;
      SPBN  A7d0;
      L     #iStep;
      L     1;
      +I    ;
      T     #iStep;
      SPA   A7d0;
A938: L     115;
      L     LW     2;
      ==I   ;
      SPB   A93a;
      SPA   A93b;
A93a: CLR   ;
      =     DIX [AR2,P#252.6];
      SET   ;
      =     DIX [AR2,P#252.7];
      U     DIX [AR2,P#10.5];
      SPBN  A7d0;
      L     #btPDIData2;
      UD    DW#16#FF;
      L     8;
      TAK   ;
      LAR1  ;
      TAK   ;
      L     DW#16#10;
      >=I   ;
      SPB   I083;
      TAK   ;
      TAR1  ;
      SLW   ;
      SPA   I084;
I083: L     DW#16#0;
I084: UD    DW#16#FFFF;
      L     #btPDIData3;
      UD    DW#16#FF;
      OW    ;
      T     #stDataEjector16.wLastFreeFlowVacuum;
      L     #iStep;
      L     1;
      +I    ;
      T     #iStep;
      SPA   A7d0;
A93b: L     116;
      L     LW     2;
      ==I   ;
      SPB   A93d;
      SPA   A93e;
A93d: CLR   ;
      =     DIX [AR2,P#252.6];
      =     DIX [AR2,P#252.7];
      U     DIX [AR2,P#10.5];
      NOT   ;
      SPBN  A7d0;
      L     #iStep;
      L     1;
      +I    ;
      T     #iStep;
      SPA   A7d0;
A93e: L     117;
      L     LW     2;
      ==I   ;
      SPB   A940;
      SPA   A941;
A940: SET   ;
      =     DIX [AR2,P#252.6];
      =     DIX [AR2,P#252.7];
      U     DIX [AR2,P#10.5];
      SPBN  A7d0;
      L     #btPDIData1;
      T     #stDataEjector16.btLeakageOfLastCycle;
      L     #btPDIData2;
      UD    DW#16#FF;
      L     8;
      TAK   ;
      LAR1  ;
      TAK   ;
      L     DW#16#10;
      >=I   ;
      SPB   I085;
      TAK   ;
      TAR1  ;
      SLW   ;
      SPA   I086;
I085: L     DW#16#0;
I086: UD    DW#16#FFFF;
      L     #btPDIData3;
      UD    DW#16#FF;
      OW    ;
      T     #stDataEjector16.wAirConsumptionOfLastCyc;
      L     #iStep;
      L     1;
      +I    ;
      T     #iStep;
      SPA   A7d0;
A941: L     118;
      L     LW     2;
      ==I   ;
      SPB   A943;
      SPA   A944;
A943: L     #iStep;
      L     1;
      +I    ;
      T     #iStep;
      SPA   A7d0;
A944: L     119;
      L     LW     2;
      ==I   ;
      SPB   A945;
      SPA   A7d0;
A945: L     0;
      T     #iStep;
A7d0: CLR   ;
      U     DIX [AR2,P#14.0];
      =     #stDataEjector1.bAirSavingFunktion_H1;
      U     DIX [AR2,P#14.1];
      =     #stDataEjector1.bPartPresent_H2;
      U     DIX [AR2,P#14.2];
      =     #stDataEjector2.bAirSavingFunktion_H1;
      U     DIX [AR2,P#14.3];
      =     #stDataEjector2.bPartPresent_H2;
      U     DIX [AR2,P#14.4];
      =     #stDataEjector3.bAirSavingFunktion_H1;
      U     DIX [AR2,P#14.5];
      =     #stDataEjector3.bPartPresent_H2;
      U     DIX [AR2,P#14.6];
      =     #stDataEjector4.bAirSavingFunktion_H1;
      U     DIX [AR2,P#14.7];
      =     #stDataEjector4.bPartPresent_H2;
      U     DIX [AR2,P#15.0];
      =     #stDataEjector5.bAirSavingFunktion_H1;
      U     DIX [AR2,P#15.1];
      =     #stDataEjector5.bPartPresent_H2;
      U     DIX [AR2,P#15.2];
      =     #stDataEjector6.bAirSavingFunktion_H1;
      U     DIX [AR2,P#15.3];
      =     #stDataEjector6.bPartPresent_H2;
      U     DIX [AR2,P#15.4];
      =     #stDataEjector7.bAirSavingFunktion_H1;
      U     DIX [AR2,P#15.5];
      =     #stDataEjector7.bPartPresent_H2;
      U     DIX [AR2,P#15.6];
      =     #stDataEjector8.bAirSavingFunktion_H1;
      U     DIX [AR2,P#15.7];
      =     #stDataEjector8.bPartPresent_H2;
      U     DIX [AR2,P#16.0];
      =     #stDataEjector9.bAirSavingFunktion_H1;
      U     DIX [AR2,P#16.1];
      =     #stDataEjector9.bPartPresent_H2;
      U     DIX [AR2,P#16.2];
      =     #stDataEjector10.bAirSavingFunktion_H1;
      U     DIX [AR2,P#16.3];
      =     #stDataEjector10.bPartPresent_H2;
      U     DIX [AR2,P#16.4];
      =     #stDataEjector11.bAirSavingFunktion_H1;
      U     DIX [AR2,P#16.5];
      =     #stDataEjector11.bPartPresent_H2;
      U     DIX [AR2,P#16.6];
      =     #stDataEjector12.bAirSavingFunktion_H1;
      U     DIX [AR2,P#16.7];
      =     #stDataEjector12.bPartPresent_H2;
      U     DIX [AR2,P#17.0];
      =     #stDataEjector13.bAirSavingFunktion_H1;
      U     DIX [AR2,P#17.1];
      =     #stDataEjector13.bPartPresent_H2;
      U     DIX [AR2,P#17.2];
      =     #stDataEjector14.bAirSavingFunktion_H1;
      U     DIX [AR2,P#17.3];
      =     #stDataEjector14.bPartPresent_H2;
      U     DIX [AR2,P#17.4];
      =     #stDataEjector15.bAirSavingFunktion_H1;
      U     DIX [AR2,P#17.5];
      =     #stDataEjector15.bPartPresent_H2;
      U     DIX [AR2,P#17.6];
      =     #stDataEjector16.bAirSavingFunktion_H1;
      U     DIX [AR2,P#17.7];
      =     #stDataEjector16.bPartPresent_H2;
      L     #iInputPressure;
      L     100;
      /I    ;
      UW    W#16#FF;
      T     #btPDOData1;
      U     DIX [AR2,P#10.6];
      NOT   ;
      =     L      0.2;
      U     DIX [AR2,P#10.7];
      NOT   ;
      U     L      0.2;
      SPBN  A947;
      SET   ;
      =     #bDeviceStateGreen;
      SPA   A948;
A947: CLR   ;
      =     #bDeviceStateGreen;
A948: CLR   ;
      U     DIX [AR2,P#10.7];
      NOT   ;
      U     DIX [AR2,P#10.6];
      SPBN  A949;
      SET   ;
      =     #bDeviceStateYellow;
      SPA   A94a;
A949: CLR   ;
      =     #bDeviceStateYellow;
A94a: CLR   ;
      U     DIX [AR2,P#10.6];
      NOT   ;
      U     DIX [AR2,P#10.7];
      SPBN  A94b;
      SET   ;
      =     #bDeviceStateOrange;
      SPA   A94c;
A94b: CLR   ;
      =     #bDeviceStateOrange;
A94c: CLR   ;
      U     DIX [AR2,P#10.6];
      U     DIX [AR2,P#10.7];
      SPBN  A94d;
      SET   ;
      =     #bDeviceStateRed;
      SPA   A94e;
A94d: CLR   ;
      =     #bDeviceStateRed;
A94e: CLR   ;
      U     DIX [AR2,P#8.0];
      SPBN  A94f;
      U     #bVacOnEjector1;
      NOT   ;
      =     DIX [AR2,P#254.0];
      U     #bBlowOffEjector1;
      =     DIX [AR2,P#254.1];
      SPA   A950;
A94f: CLR   ;
      U     #bVacOnEjector1;
      =     DIX [AR2,P#254.0];
      U     #bBlowOffEjector1;
      =     DIX [AR2,P#254.1];
A950: CLR   ;
      U     DIX [AR2,P#8.1];
      SPBN  A951;
      U     #bVacOnEjector2;
      NOT   ;
      =     DIX [AR2,P#254.2];
      U     #bBlowOffEjector2;
      =     DIX [AR2,P#254.3];
      SPA   A952;
A951: CLR   ;
      U     #bVacOnEjector2;
      =     DIX [AR2,P#254.2];
      U     #bBlowOffEjector2;
      =     DIX [AR2,P#254.3];
A952: CLR   ;
      U     DIX [AR2,P#8.2];
      SPBN  A953;
      U     #bVacOnEjector3;
      NOT   ;
      =     DIX [AR2,P#254.4];
      U     #bBlowOffEjector3;
      =     DIX [AR2,P#254.5];
      SPA   A954;
A953: CLR   ;
      U     #bVacOnEjector3;
      =     DIX [AR2,P#254.4];
      U     #bBlowOffEjector3;
      =     DIX [AR2,P#254.5];
A954: CLR   ;
      U     DIX [AR2,P#8.3];
      SPBN  A955;
      U     #bVacOnEjector4;
      NOT   ;
      =     DIX [AR2,P#254.6];
      U     #bBlowOffEjector4;
      =     DIX [AR2,P#254.7];
      SPA   A956;
A955: CLR   ;
      U     #bVacOnEjector4;
      =     DIX [AR2,P#254.6];
      U     #bBlowOffEjector4;
      =     DIX [AR2,P#254.7];
A956: CLR   ;
      U     DIX [AR2,P#8.4];
      SPBN  A957;
      U     #bVacOnEjector5;
      NOT   ;
      =     DIX [AR2,P#255.0];
      U     #bBlowOffEjector5;
      =     DIX [AR2,P#255.1];
      SPA   A958;
A957: CLR   ;
      U     #bVacOnEjector5;
      =     DIX [AR2,P#255.0];
      U     #bBlowOffEjector5;
      =     DIX [AR2,P#255.1];
A958: CLR   ;
      U     DIX [AR2,P#8.5];
      SPBN  A959;
      U     #bVacOnEjector6;
      NOT   ;
      =     DIX [AR2,P#255.2];
      U     #bBlowOffEjector6;
      =     DIX [AR2,P#255.3];
      SPA   A95a;
A959: CLR   ;
      U     #bVacOnEjector6;
      =     DIX [AR2,P#255.2];
      U     #bBlowOffEjector6;
      =     DIX [AR2,P#255.3];
A95a: CLR   ;
      U     DIX [AR2,P#8.6];
      SPBN  A95b;
      U     #bVacOnEjector7;
      NOT   ;
      =     DIX [AR2,P#255.4];
      U     #bBlowOffEjector7;
      =     DIX [AR2,P#255.5];
      SPA   A95c;
A95b: CLR   ;
      U     #bVacOnEjector7;
      =     DIX [AR2,P#255.4];
      U     #bBlowOffEjector7;
      =     DIX [AR2,P#255.5];
A95c: CLR   ;
      U     DIX [AR2,P#8.7];
      SPBN  A95d;
      U     #bVacOnEjector8;
      NOT   ;
      =     DIX [AR2,P#255.6];
      U     #bBlowOffEjector8;
      =     DIX [AR2,P#255.7];
      SPA   A95e;
A95d: CLR   ;
      U     #bVacOnEjector8;
      =     DIX [AR2,P#255.6];
      U     #bBlowOffEjector8;
      =     DIX [AR2,P#255.7];
A95e: CLR   ;
      U     DIX [AR2,P#9.0];
      SPBN  A95f;
      U     #bVacOnEjector9;
      NOT   ;
      =     DIX [AR2,P#256.0];
      U     #bBlowOffEjector9;
      =     DIX [AR2,P#256.1];
      SPA   A960;
A95f: CLR   ;
      U     #bVacOnEjector9;
      =     DIX [AR2,P#256.0];
      U     #bBlowOffEjector9;
      =     DIX [AR2,P#256.1];
A960: CLR   ;
      U     DIX [AR2,P#9.1];
      SPBN  A961;
      U     #bVacOnEjector10;
      NOT   ;
      =     DIX [AR2,P#256.2];
      U     #bBlowOffEjector10;
      =     DIX [AR2,P#256.3];
      SPA   A962;
A961: CLR   ;
      U     #bVacOnEjector10;
      =     DIX [AR2,P#256.2];
      U     #bBlowOffEjector10;
      =     DIX [AR2,P#256.3];
A962: CLR   ;
      U     DIX [AR2,P#9.2];
      SPBN  A963;
      U     #bVacOnEjector11;
      NOT   ;
      =     DIX [AR2,P#256.4];
      U     #bBlowOffEjector11;
      =     DIX [AR2,P#256.5];
      SPA   A964;
A963: CLR   ;
      U     #bVacOnEjector11;
      =     DIX [AR2,P#256.4];
      U     #bBlowOffEjector11;
      =     DIX [AR2,P#256.5];
A964: CLR   ;
      U     DIX [AR2,P#9.3];
      SPBN  A965;
      U     #bVacOnEjector12;
      NOT   ;
      =     DIX [AR2,P#256.6];
      U     #bBlowOffEjector12;
      =     DIX [AR2,P#256.7];
      SPA   A966;
A965: CLR   ;
      U     #bVacOnEjector12;
      =     DIX [AR2,P#256.6];
      U     #bBlowOffEjector12;
      =     DIX [AR2,P#256.7];
A966: CLR   ;
      U     DIX [AR2,P#9.4];
      SPBN  A967;
      U     #bVacOnEjector13;
      NOT   ;
      =     DIX [AR2,P#257.0];
      U     #bBlowOffEjector13;
      =     DIX [AR2,P#257.1];
      SPA   A968;
A967: CLR   ;
      U     #bVacOnEjector13;
      =     DIX [AR2,P#257.0];
      U     #bBlowOffEjector13;
      =     DIX [AR2,P#257.1];
A968: CLR   ;
      U     DIX [AR2,P#9.5];
      SPBN  A969;
      U     #bVacOnEjector14;
      NOT   ;
      =     DIX [AR2,P#257.2];
      U     #bBlowOffEjector14;
      =     DIX [AR2,P#257.3];
      SPA   A96a;
A969: CLR   ;
      U     #bVacOnEjector14;
      =     DIX [AR2,P#257.2];
      U     #bBlowOffEjector14;
      =     DIX [AR2,P#257.3];
A96a: CLR   ;
      U     DIX [AR2,P#9.6];
      SPBN  A96b;
      U     #bVacOnEjector15;
      NOT   ;
      =     DIX [AR2,P#257.4];
      U     #bBlowOffEjector15;
      =     DIX [AR2,P#257.5];
      SPA   A96c;
A96b: CLR   ;
      U     #bVacOnEjector15;
      =     DIX [AR2,P#257.4];
      U     #bBlowOffEjector15;
      =     DIX [AR2,P#257.5];
A96c: CLR   ;
      U     DIX [AR2,P#9.7];
      SPBN  A96d;
      U     #bVacOnEjector16;
      NOT   ;
      =     DIX [AR2,P#257.6];
      U     #bBlowOffEjector16;
      =     DIX [AR2,P#257.7];
      SPA   A96e;
A96d: CLR   ;
      U     #bVacOnEjector16;
      =     DIX [AR2,P#257.6];
      U     #bBlowOffEjector16;
      =     DIX [AR2,P#257.7];
A96e: CLR   ;
      U     L      0.1;
      SAVE  ;
      BE    ;
END_FUNCTION_BLOCK

